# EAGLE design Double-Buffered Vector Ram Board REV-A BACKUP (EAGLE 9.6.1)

## Sheet 1 of 4: Vector Ram Control
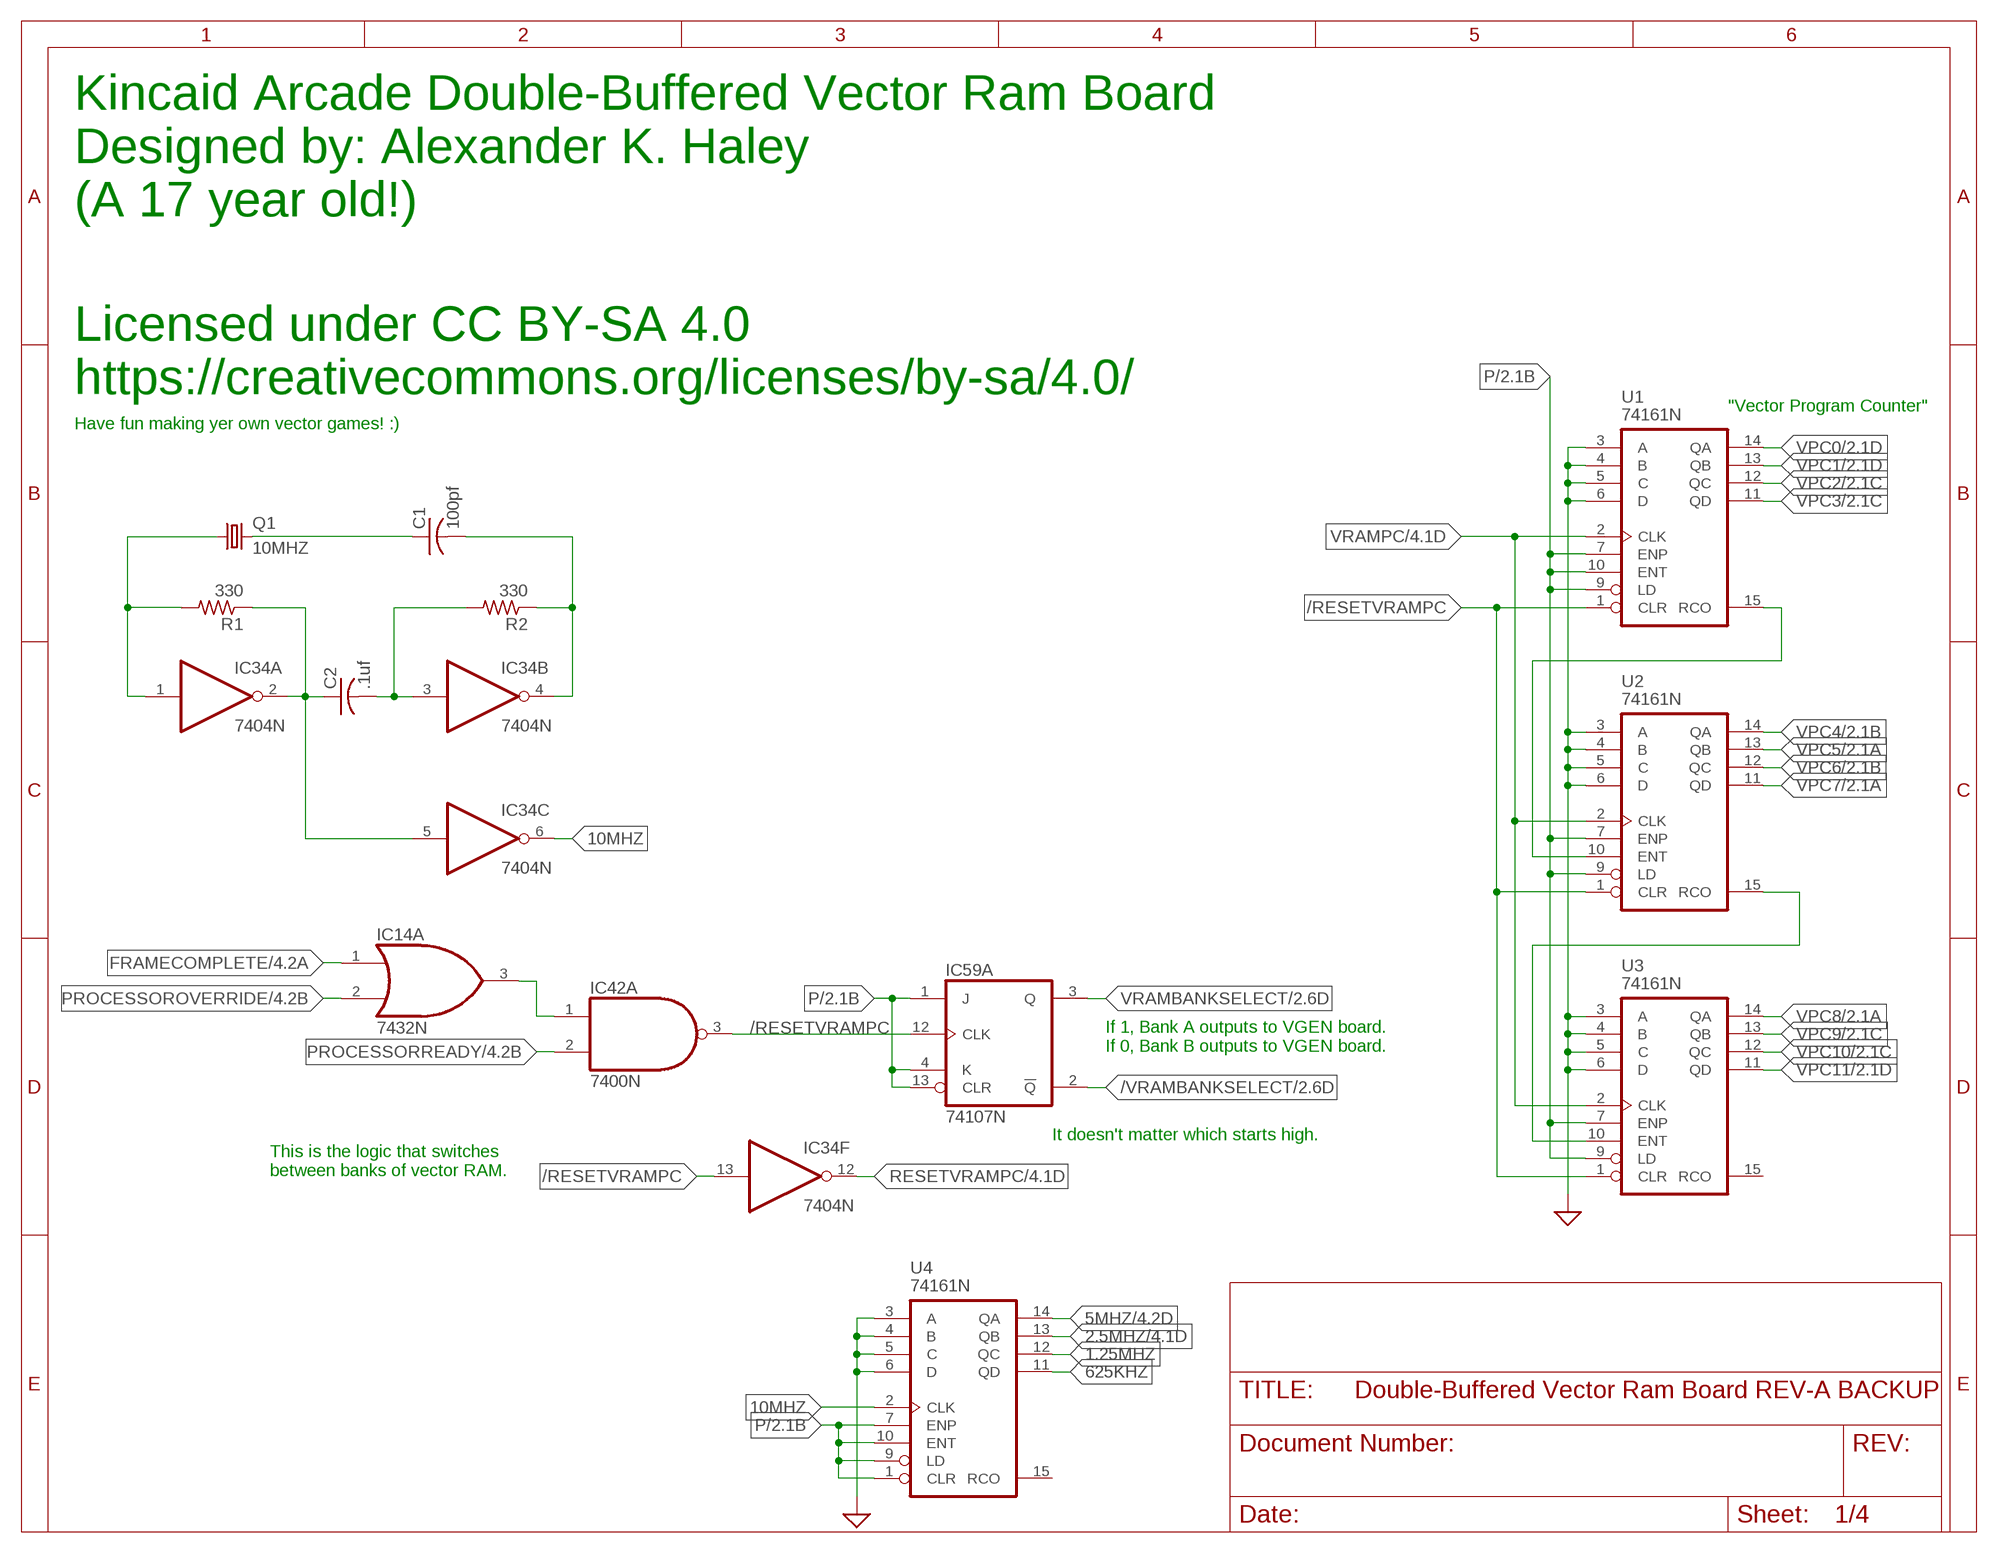
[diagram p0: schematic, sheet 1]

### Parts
C1  100pf  C-US025-030X050  [C025-030X050]
C2  .1uf  C-US050-050X075  [C050-050X075]
IC14  7432N  [DIL14]
IC34  7404N  [DIL14]
IC42  7400N  [DIL14]
IC59  74107N  [DIL14]
Q1  10MHZ  CRYSTALHC49S  [HC49/S]
R1  330  R-US_0207/10  [0207/10]
R2  330  R-US_0207/10  [0207/10]
U1  74161N  [DIL16]
U2  74161N  [DIL16]
U3  74161N  [DIL16]
U4  74161N  [DIL16]

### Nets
1.25MHZ: U4.12(QC)
2.5MHZ: U4.13(QB) ; also sheet 4
5MHZ: U4.14(QA) ; also sheet 4
10MHZ: IC34.6(C:O) U4.2(CLK)
625KHZ: U4.11(QD)
/RESETVRAMPC: IC34.13(F:I) IC42.3(A:O) IC59.12(A:CLK) U1.1(CLR) U2.1(CLR) U3.1(CLR)
/VRAMBANKSELECT: IC59.2(A:!Q) ; also sheet 2,3
FRAMECOMPLETE: IC14.1(A:I0) ; also sheet 4
GND: U1.3(A) U1.4(B) U1.5(C) U1.6(D) U2.3(A) U2.4(B) U2.5(C) U2.6(D) U3.3(A) U3.4(B) U3.5(C) U3.6(D) U4.3(A) U4.4(B) U4.5(C) U4.6(D) ; supply symbol labelled SUP ; also sheet 2,3,4
N$2: IC14.3(A:O) IC42.1(A:I0)
N$5: U2.15(RCO) U3.10(ENT)
N$6: U1.15(RCO) U2.10(ENT)
N$48: IC34.1(A:I) Q1.1 R1.2
N$52: C2.1 IC34.2(A:O) IC34.5(C:I) R1.1
N$61: C2.2 IC34.3(B:I) R2.2
N$69: C1.1 Q1.2
N$74: C1.2 IC34.4(B:O) R2.1
P: IC59.1(A:J) IC59.4(A:K) IC59.13(A:CLR) U1.7(ENP) U1.9(LD) U1.10(ENT) U2.7(ENP) U2.9(LD) U3.7(ENP) U3.9(LD) U4.1(CLR) U4.7(ENP) U4.9(LD) U4.10(ENT) ; also sheet 2,3,4
PROCESSOROVERRIDE: IC14.2(A:I1) ; also sheet 4
PROCESSORREADY: IC42.2(A:I1) ; also sheet 4
RESETVRAMPC: IC34.12(F:O) ; also sheet 4
VPC0: U1.14(QA) ; also sheet 2,3
VPC1: U1.13(QB) ; also sheet 2,3
VPC2: U1.12(QC) ; also sheet 2,3
VPC3: U1.11(QD) ; also sheet 2,3
VPC4: U2.14(QA) ; also sheet 2,3
VPC5: U2.13(QB) ; also sheet 2,3
VPC6: U2.12(QC) ; also sheet 2,3
VPC7: U2.11(QD) ; also sheet 2,3
VPC8: U3.14(QA) ; also sheet 2,3
VPC9: U3.13(QB) ; also sheet 2,3
VPC10: U3.12(QC) ; also sheet 2,3
VPC11: U3.11(QD) ; also sheet 2,3
VRAMBANKSELECT: IC59.3(A:Q) ; also sheet 2,3
VRAMPC: U1.2(CLK) U2.2(CLK) U3.2(CLK) ; also sheet 4
Unconnected: U3.15(RCO) U4.15(RCO)

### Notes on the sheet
- Kincaid Arcade Double-Buffered Vector Ram Board
- Designed by: Alexander K. Haley
- (A 17 year old!)
- Licensed under CC BY-SA 4.0
- https://creativecommons.org/licenses/by-sa/4.0/
- "Vector Program Counter"
- Have fun making yer own vector games! :)
- If 1, Bank A outputs to VGEN board.
  If 0, Bank B outputs to VGEN board.
- It doesn't matter which starts high.
- This is the logic that switches 
  between banks of vector RAM.

## Sheet 2 of 4: Vector Ram Bank A
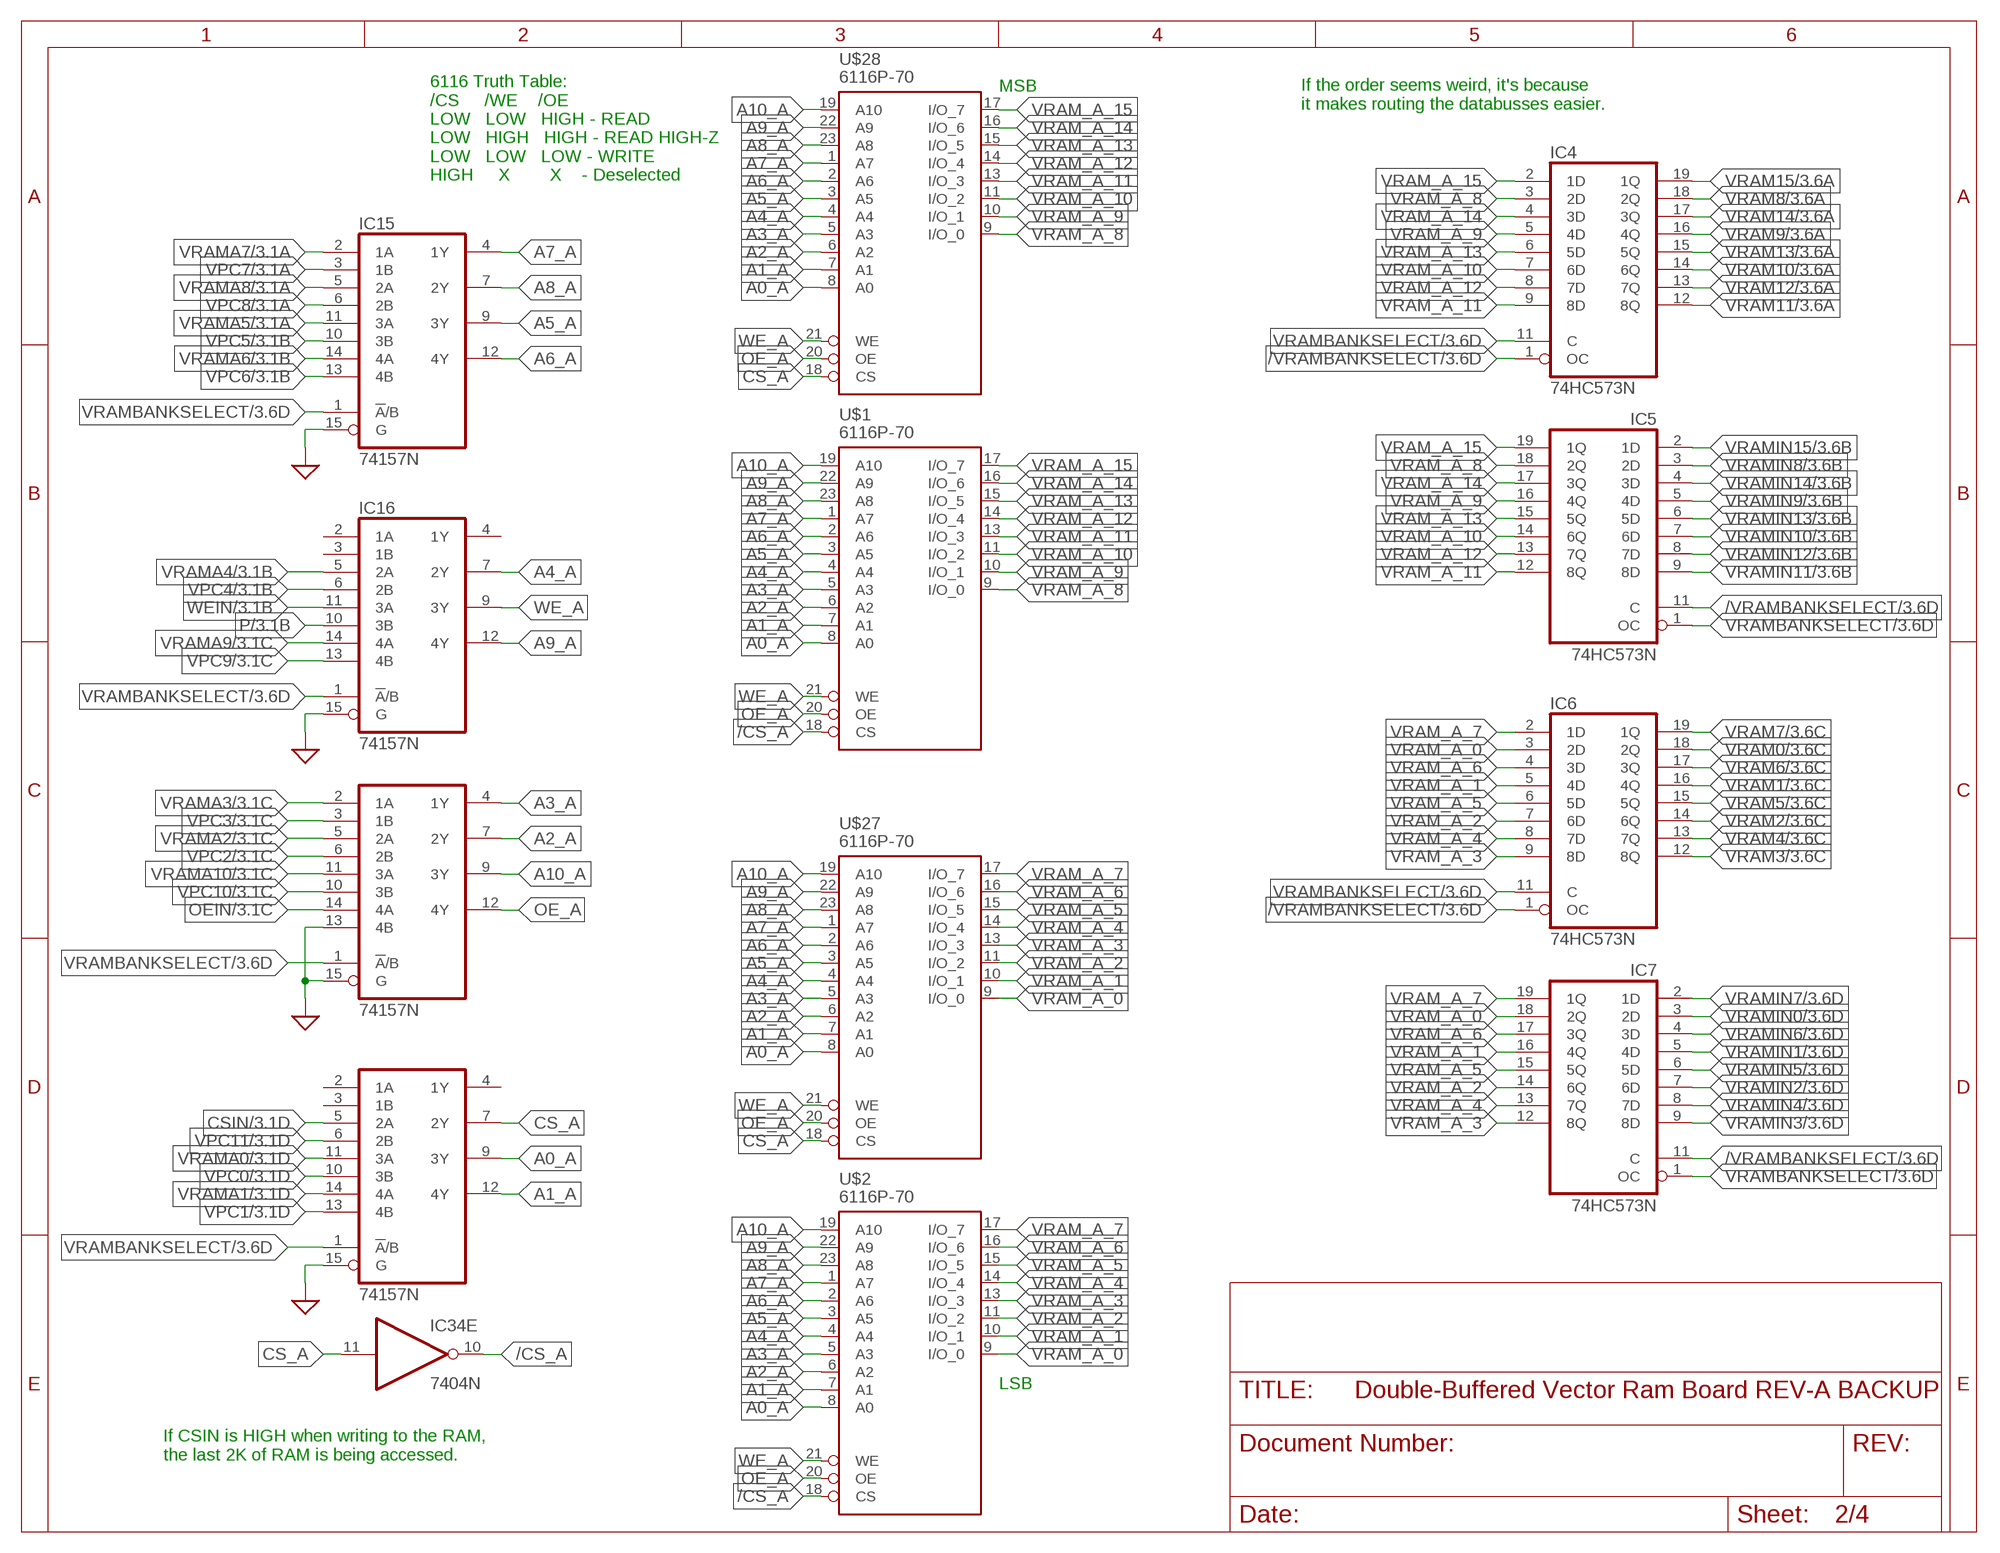
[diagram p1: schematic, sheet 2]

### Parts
IC4  74HC573N  [DIL20]
IC5  74HC573N  [DIL20]
IC6  74HC573N  [DIL20]
IC7  74HC573N  [DIL20]
IC15  74157N  [DIL16]
IC16  74157N  [DIL16]
IC17  74157N  [DIL16]
IC18  74157N  [DIL16]
U$1  6116P-70  DS1220AB/AD  [DIL24]
U$2  6116P-70  DS1220AB/AD  [DIL24]
U$27  6116P-70  [DIL24]
U$28  6116P-70  [DIL24]

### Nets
/CS_A: IC34.10(E:O) U$1.18(CS) U$2.18(CS)
/VRAMBANKSELECT: IC4.1(OC) IC5.11(C) IC6.1(OC) IC7.11(C) ; also sheet 1,3
A0_A: IC18.9(3Y) U$1.8(A0) U$2.8(A0) U$27.8(A0) U$28.8(A0)
A1_A: IC18.12(4Y) U$1.7(A1) U$2.7(A1) U$27.7(A1) U$28.7(A1)
A2_A: IC17.7(2Y) U$1.6(A2) U$2.6(A2) U$27.6(A2) U$28.6(A2)
A3_A: IC17.4(1Y) U$1.5(A3) U$2.5(A3) U$27.5(A3) U$28.5(A3)
A4_A: IC16.7(2Y) U$1.4(A4) U$2.4(A4) U$27.4(A4) U$28.4(A4)
A5_A: IC15.9(3Y) U$1.3(A5) U$2.3(A5) U$27.3(A5) U$28.3(A5)
A6_A: IC15.12(4Y) U$1.2(A6) U$2.2(A6) U$27.2(A6) U$28.2(A6)
A7_A: IC15.4(1Y) U$1.1(A7) U$2.1(A7) U$27.1(A7) U$28.1(A7)
A8_A: IC15.7(2Y) U$1.23(A8) U$2.23(A8) U$27.23(A8) U$28.23(A8)
A9_A: IC16.12(4Y) U$1.22(A9) U$2.22(A9) U$27.22(A9) U$28.22(A9)
A10_A: IC17.9(3Y) U$1.19(A10) U$2.19(A10) U$27.19(A10) U$28.19(A10)
CS_A: IC18.7(2Y) IC34.11(E:I) U$27.18(CS) U$28.18(CS)
CSIN: IC18.5(2A) ; also sheet 3,4
GND: IC15.15(G) IC16.15(G) IC17.13(4B) IC17.15(G) IC18.15(G) ; supply symbol labelled SUP ; also sheet 1,3,4
OE_A: IC17.12(4Y) U$1.20(OE) U$2.20(OE) U$27.20(OE) U$28.20(OE)
OEIN: IC17.14(4A) ; also sheet 3,4
P: IC16.10(3B) ; also sheet 1,3,4
VPC0: IC18.10(3B) ; also sheet 1,3
VPC1: IC18.13(4B) ; also sheet 1,3
VPC2: IC17.6(2B) ; also sheet 1,3
VPC3: IC17.3(1B) ; also sheet 1,3
VPC4: IC16.6(2B) ; also sheet 1,3
VPC5: IC15.10(3B) ; also sheet 1,3
VPC6: IC15.13(4B) ; also sheet 1,3
VPC7: IC15.3(1B) ; also sheet 1,3
VPC8: IC15.6(2B) ; also sheet 1,3
VPC9: IC16.13(4B) ; also sheet 1,3
VPC10: IC17.10(3B) ; also sheet 1,3
VPC11: IC18.6(2B) ; also sheet 1,3
VRAM0: IC6.18(2Q) ; also sheet 3,4
VRAM1: IC6.16(4Q) ; also sheet 3,4
VRAM2: IC6.14(6Q) ; also sheet 3,4
VRAM3: IC6.12(8Q) ; also sheet 3,4
VRAM4: IC6.13(7Q) ; also sheet 3,4
VRAM5: IC6.15(5Q) ; also sheet 3,4
VRAM6: IC6.17(3Q) ; also sheet 3,4
VRAM7: IC6.19(1Q) ; also sheet 3,4
VRAM8: IC4.18(2Q) ; also sheet 3,4
VRAM9: IC4.16(4Q) ; also sheet 3,4
VRAM10: IC4.14(6Q) ; also sheet 3,4
VRAM11: IC4.12(8Q) ; also sheet 3,4
VRAM12: IC4.13(7Q) ; also sheet 3,4
VRAM13: IC4.15(5Q) ; also sheet 3,4
VRAM14: IC4.17(3Q) ; also sheet 3,4
VRAM15: IC4.19(1Q) ; also sheet 3,4
VRAM_A_0: IC6.3(2D) IC7.18(2Q) U$2.9(I/O_0) U$27.9(I/O_0)
VRAM_A_1: IC6.5(4D) IC7.16(4Q) U$2.10(I/O_1) U$27.10(I/O_1)
VRAM_A_2: IC6.7(6D) IC7.14(6Q) U$2.11(I/O_2) U$27.11(I/O_2)
VRAM_A_3: IC6.9(8D) IC7.12(8Q) U$2.13(I/O_3) U$27.13(I/O_3)
VRAM_A_4: IC6.8(7D) IC7.13(7Q) U$2.14(I/O_4) U$27.14(I/O_4)
VRAM_A_5: IC6.6(5D) IC7.15(5Q) U$2.15(I/O_5) U$27.15(I/O_5)
VRAM_A_6: IC6.4(3D) IC7.17(3Q) U$2.16(I/O_6) U$27.16(I/O_6)
VRAM_A_7: IC6.2(1D) IC7.19(1Q) U$2.17(I/O_7) U$27.17(I/O_7)
VRAM_A_8: IC4.3(2D) IC5.18(2Q) U$1.9(I/O_0) U$28.9(I/O_0)
VRAM_A_9: IC4.5(4D) IC5.16(4Q) U$1.10(I/O_1) U$28.10(I/O_1)
VRAM_A_10: IC4.7(6D) IC5.14(6Q) U$1.11(I/O_2) U$28.11(I/O_2)
VRAM_A_11: IC4.9(8D) IC5.12(8Q) U$1.13(I/O_3) U$28.13(I/O_3)
VRAM_A_12: IC4.8(7D) IC5.13(7Q) U$1.14(I/O_4) U$28.14(I/O_4)
VRAM_A_13: IC4.6(5D) IC5.15(5Q) U$1.15(I/O_5) U$28.15(I/O_5)
VRAM_A_14: IC4.4(3D) IC5.17(3Q) U$1.16(I/O_6) U$28.16(I/O_6)
VRAM_A_15: IC4.2(1D) IC5.19(1Q) U$1.17(I/O_7) U$28.17(I/O_7)
VRAMA0: IC18.11(3A) ; also sheet 3,4
VRAMA1: IC18.14(4A) ; also sheet 3,4
VRAMA2: IC17.5(2A) ; also sheet 3,4
VRAMA3: IC17.2(1A) ; also sheet 3,4
VRAMA4: IC16.5(2A) ; also sheet 3,4
VRAMA5: IC15.11(3A) ; also sheet 3,4
VRAMA6: IC15.14(4A) ; also sheet 3,4
VRAMA7: IC15.2(1A) ; also sheet 3,4
VRAMA8: IC15.5(2A) ; also sheet 3,4
VRAMA9: IC16.14(4A) ; also sheet 3,4
VRAMA10: IC17.11(3A) ; also sheet 3,4
VRAMBANKSELECT: IC4.11(C) IC5.1(OC) IC6.11(C) IC7.1(OC) IC15.1(!A!/B) IC16.1(!A!/B) IC17.1(!A!/B) IC18.1(!A!/B) ; also sheet 1,3
VRAMIN0: IC7.3(2D) ; also sheet 3,4
VRAMIN1: IC7.5(4D) ; also sheet 3,4
VRAMIN2: IC7.7(6D) ; also sheet 3,4
VRAMIN3: IC7.9(8D) ; also sheet 3,4
VRAMIN4: IC7.8(7D) ; also sheet 3,4
VRAMIN5: IC7.6(5D) ; also sheet 3,4
VRAMIN6: IC7.4(3D) ; also sheet 3,4
VRAMIN7: IC7.2(1D) ; also sheet 3,4
VRAMIN8: IC5.3(2D) ; also sheet 3,4
VRAMIN9: IC5.5(4D) ; also sheet 3,4
VRAMIN10: IC5.7(6D) ; also sheet 3,4
VRAMIN11: IC5.9(8D) ; also sheet 3,4
VRAMIN12: IC5.8(7D) ; also sheet 3,4
VRAMIN13: IC5.6(5D) ; also sheet 3,4
VRAMIN14: IC5.4(3D) ; also sheet 3,4
VRAMIN15: IC5.2(1D) ; also sheet 3,4
WE_A: IC16.9(3Y) U$1.21(WE) U$2.21(WE) U$27.21(WE) U$28.21(WE)
WEIN: IC16.11(3A) ; also sheet 3,4
Unconnected: IC16.2(1A) IC16.3(1B) IC16.4(1Y) IC18.2(1A) IC18.3(1B) IC18.4(1Y)

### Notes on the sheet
- MSB
- If the order seems weird, it's because
  it makes routing the databusses easier.
- 6116 Truth Table:
  /CS     /WE    /OE
  LOW   LOW   HIGH - READ
  LOW   HIGH   HIGH - READ HIGH-Z
  LOW   LOW   LOW - WRITE
  HIGH     X        X    - Deselected
- LSB
- If CSIN is HIGH when writing to the RAM, 
  the last 2K of RAM is being accessed.

## Sheet 3 of 4: Vector Ram Bank B
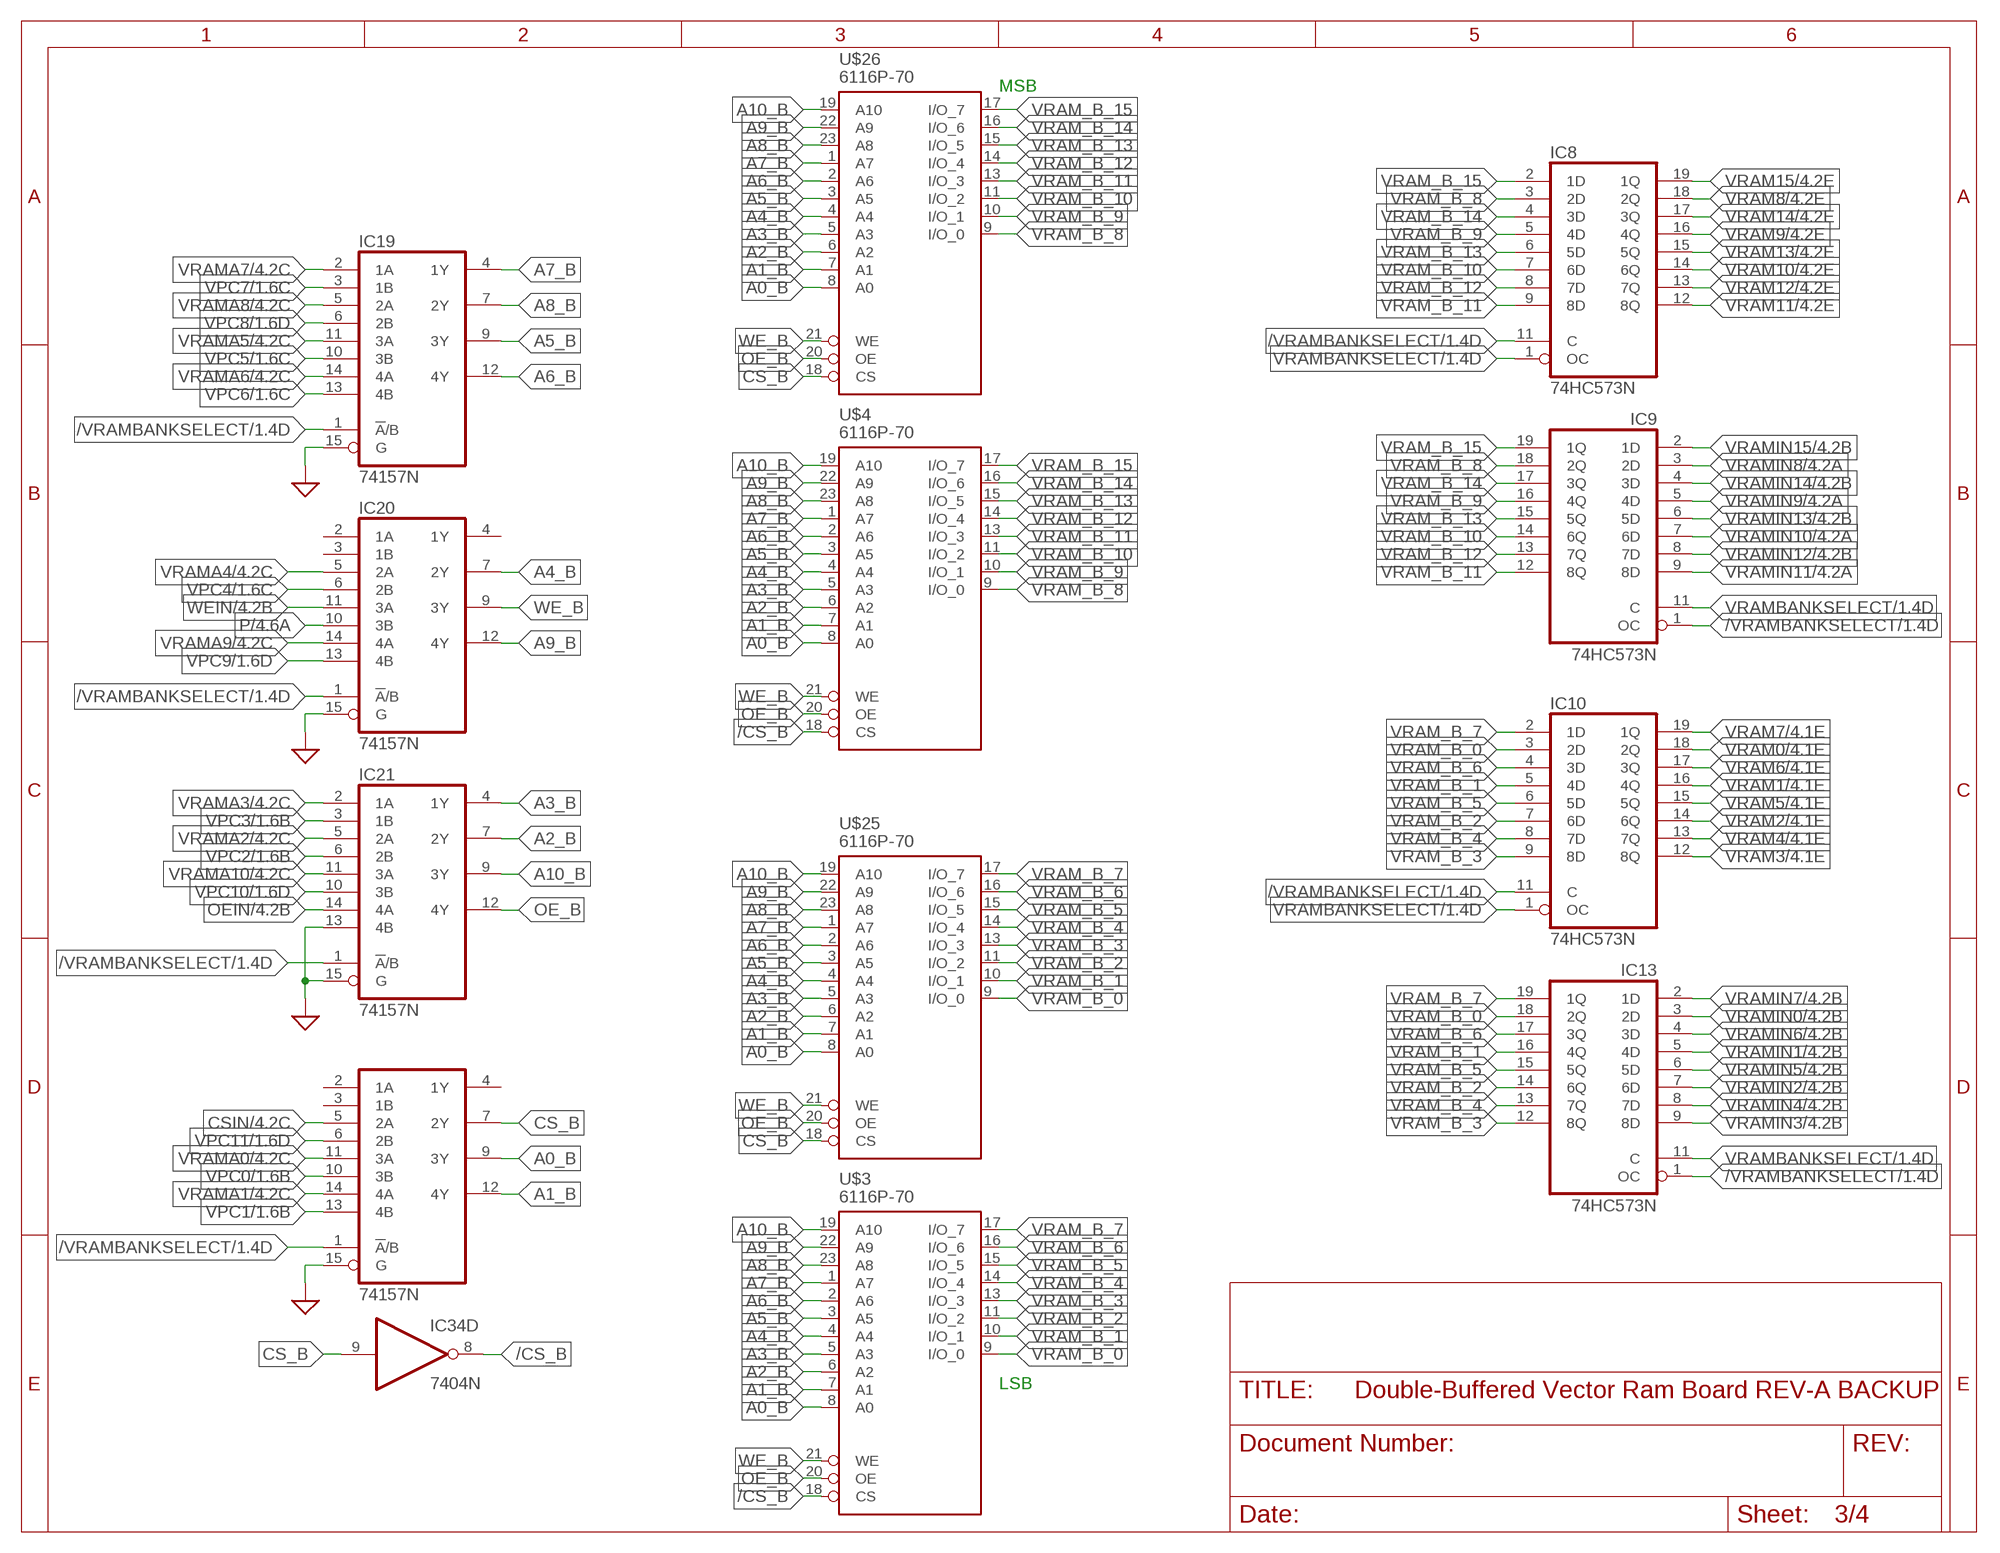
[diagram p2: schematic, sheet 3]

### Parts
IC8  74HC573N  [DIL20]
IC9  74HC573N  [DIL20]
IC10  74HC573N  [DIL20]
IC13  74HC573N  [DIL20]
IC19  74157N  [DIL16]
IC20  74157N  [DIL16]
IC21  74157N  [DIL16]
IC22  74157N  [DIL16]
U$3  6116P-70  DS1220AB/AD  [DIL24]
U$4  6116P-70  DS1220AB/AD  [DIL24]
U$25  6116P-70  [DIL24]
U$26  6116P-70  [DIL24]

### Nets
/CS_B: IC34.8(D:O) U$3.18(CS) U$4.18(CS)
/VRAMBANKSELECT: IC8.11(C) IC9.1(OC) IC10.11(C) IC13.1(OC) IC19.1(!A!/B) IC20.1(!A!/B) IC21.1(!A!/B) IC22.1(!A!/B) ; also sheet 1,2
A0_B: IC22.9(3Y) U$3.8(A0) U$4.8(A0) U$25.8(A0) U$26.8(A0)
A1_B: IC22.12(4Y) U$3.7(A1) U$4.7(A1) U$25.7(A1) U$26.7(A1)
A2_B: IC21.7(2Y) U$3.6(A2) U$4.6(A2) U$25.6(A2) U$26.6(A2)
A3_B: IC21.4(1Y) U$3.5(A3) U$4.5(A3) U$25.5(A3) U$26.5(A3)
A4_B: IC20.7(2Y) U$3.4(A4) U$4.4(A4) U$25.4(A4) U$26.4(A4)
A5_B: IC19.9(3Y) U$3.3(A5) U$4.3(A5) U$25.3(A5) U$26.3(A5)
A6_B: IC19.12(4Y) U$3.2(A6) U$4.2(A6) U$25.2(A6) U$26.2(A6)
A7_B: IC19.4(1Y) U$3.1(A7) U$4.1(A7) U$25.1(A7) U$26.1(A7)
A8_B: IC19.7(2Y) U$3.23(A8) U$4.23(A8) U$25.23(A8) U$26.23(A8)
A9_B: IC20.12(4Y) U$3.22(A9) U$4.22(A9) U$25.22(A9) U$26.22(A9)
A10_B: IC21.9(3Y) U$3.19(A10) U$4.19(A10) U$25.19(A10) U$26.19(A10)
CS_B: IC22.7(2Y) IC34.9(D:I) U$25.18(CS) U$26.18(CS)
CSIN: IC22.5(2A) ; also sheet 2,4
GND: IC19.15(G) IC20.15(G) IC21.13(4B) IC21.15(G) IC22.15(G) ; supply symbol labelled SUP ; also sheet 1,2,4
OE_B: IC21.12(4Y) U$3.20(OE) U$4.20(OE) U$25.20(OE) U$26.20(OE)
OEIN: IC21.14(4A) ; also sheet 2,4
P: IC20.10(3B) ; also sheet 1,2,4
VPC0: IC22.10(3B) ; also sheet 1,2
VPC1: IC22.13(4B) ; also sheet 1,2
VPC2: IC21.6(2B) ; also sheet 1,2
VPC3: IC21.3(1B) ; also sheet 1,2
VPC4: IC20.6(2B) ; also sheet 1,2
VPC5: IC19.10(3B) ; also sheet 1,2
VPC6: IC19.13(4B) ; also sheet 1,2
VPC7: IC19.3(1B) ; also sheet 1,2
VPC8: IC19.6(2B) ; also sheet 1,2
VPC9: IC20.13(4B) ; also sheet 1,2
VPC10: IC21.10(3B) ; also sheet 1,2
VPC11: IC22.6(2B) ; also sheet 1,2
VRAM0: IC10.18(2Q) ; also sheet 2,4
VRAM1: IC10.16(4Q) ; also sheet 2,4
VRAM2: IC10.14(6Q) ; also sheet 2,4
VRAM3: IC10.12(8Q) ; also sheet 2,4
VRAM4: IC10.13(7Q) ; also sheet 2,4
VRAM5: IC10.15(5Q) ; also sheet 2,4
VRAM6: IC10.17(3Q) ; also sheet 2,4
VRAM7: IC10.19(1Q) ; also sheet 2,4
VRAM8: IC8.18(2Q) ; also sheet 2,4
VRAM9: IC8.16(4Q) ; also sheet 2,4
VRAM10: IC8.14(6Q) ; also sheet 2,4
VRAM11: IC8.12(8Q) ; also sheet 2,4
VRAM12: IC8.13(7Q) ; also sheet 2,4
VRAM13: IC8.15(5Q) ; also sheet 2,4
VRAM14: IC8.17(3Q) ; also sheet 2,4
VRAM15: IC8.19(1Q) ; also sheet 2,4
VRAM_B_0: IC10.3(2D) IC13.18(2Q) U$3.9(I/O_0) U$25.9(I/O_0)
VRAM_B_1: IC10.5(4D) IC13.16(4Q) U$3.10(I/O_1) U$25.10(I/O_1)
VRAM_B_2: IC10.7(6D) IC13.14(6Q) U$3.11(I/O_2) U$25.11(I/O_2)
VRAM_B_3: IC10.9(8D) IC13.12(8Q) U$3.13(I/O_3) U$25.13(I/O_3)
VRAM_B_4: IC10.8(7D) IC13.13(7Q) U$3.14(I/O_4) U$25.14(I/O_4)
VRAM_B_5: IC10.6(5D) IC13.15(5Q) U$3.15(I/O_5) U$25.15(I/O_5)
VRAM_B_6: IC10.4(3D) IC13.17(3Q) U$3.16(I/O_6) U$25.16(I/O_6)
VRAM_B_7: IC10.2(1D) IC13.19(1Q) U$3.17(I/O_7) U$25.17(I/O_7)
VRAM_B_8: IC8.3(2D) IC9.18(2Q) U$4.9(I/O_0) U$26.9(I/O_0)
VRAM_B_9: IC8.5(4D) IC9.16(4Q) U$4.10(I/O_1) U$26.10(I/O_1)
VRAM_B_10: IC8.7(6D) IC9.14(6Q) U$4.11(I/O_2) U$26.11(I/O_2)
VRAM_B_11: IC8.9(8D) IC9.12(8Q) U$4.13(I/O_3) U$26.13(I/O_3)
VRAM_B_12: IC8.8(7D) IC9.13(7Q) U$4.14(I/O_4) U$26.14(I/O_4)
VRAM_B_13: IC8.6(5D) IC9.15(5Q) U$4.15(I/O_5) U$26.15(I/O_5)
VRAM_B_14: IC8.4(3D) IC9.17(3Q) U$4.16(I/O_6) U$26.16(I/O_6)
VRAM_B_15: IC8.2(1D) IC9.19(1Q) U$4.17(I/O_7) U$26.17(I/O_7)
VRAMA0: IC22.11(3A) ; also sheet 2,4
VRAMA1: IC22.14(4A) ; also sheet 2,4
VRAMA2: IC21.5(2A) ; also sheet 2,4
VRAMA3: IC21.2(1A) ; also sheet 2,4
VRAMA4: IC20.5(2A) ; also sheet 2,4
VRAMA5: IC19.11(3A) ; also sheet 2,4
VRAMA6: IC19.14(4A) ; also sheet 2,4
VRAMA7: IC19.2(1A) ; also sheet 2,4
VRAMA8: IC19.5(2A) ; also sheet 2,4
VRAMA9: IC20.14(4A) ; also sheet 2,4
VRAMA10: IC21.11(3A) ; also sheet 2,4
VRAMBANKSELECT: IC8.1(OC) IC9.11(C) IC10.1(OC) IC13.11(C) ; also sheet 1,2
VRAMIN0: IC13.3(2D) ; also sheet 2,4
VRAMIN1: IC13.5(4D) ; also sheet 2,4
VRAMIN2: IC13.7(6D) ; also sheet 2,4
VRAMIN3: IC13.9(8D) ; also sheet 2,4
VRAMIN4: IC13.8(7D) ; also sheet 2,4
VRAMIN5: IC13.6(5D) ; also sheet 2,4
VRAMIN6: IC13.4(3D) ; also sheet 2,4
VRAMIN7: IC13.2(1D) ; also sheet 2,4
VRAMIN8: IC9.3(2D) ; also sheet 2,4
VRAMIN9: IC9.5(4D) ; also sheet 2,4
VRAMIN10: IC9.7(6D) ; also sheet 2,4
VRAMIN11: IC9.9(8D) ; also sheet 2,4
VRAMIN12: IC9.8(7D) ; also sheet 2,4
VRAMIN13: IC9.6(5D) ; also sheet 2,4
VRAMIN14: IC9.4(3D) ; also sheet 2,4
VRAMIN15: IC9.2(1D) ; also sheet 2,4
WE_B: IC20.9(3Y) U$3.21(WE) U$4.21(WE) U$25.21(WE) U$26.21(WE)
WEIN: IC20.11(3A) ; also sheet 2,4
Unconnected: IC20.2(1A) IC20.3(1B) IC20.4(1Y) IC22.2(1A) IC22.3(1B) IC22.4(1Y)

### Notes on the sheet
- MSB
- LSB

## Sheet 4 of 4: Connectors, Pullups, and Filter Capacitors
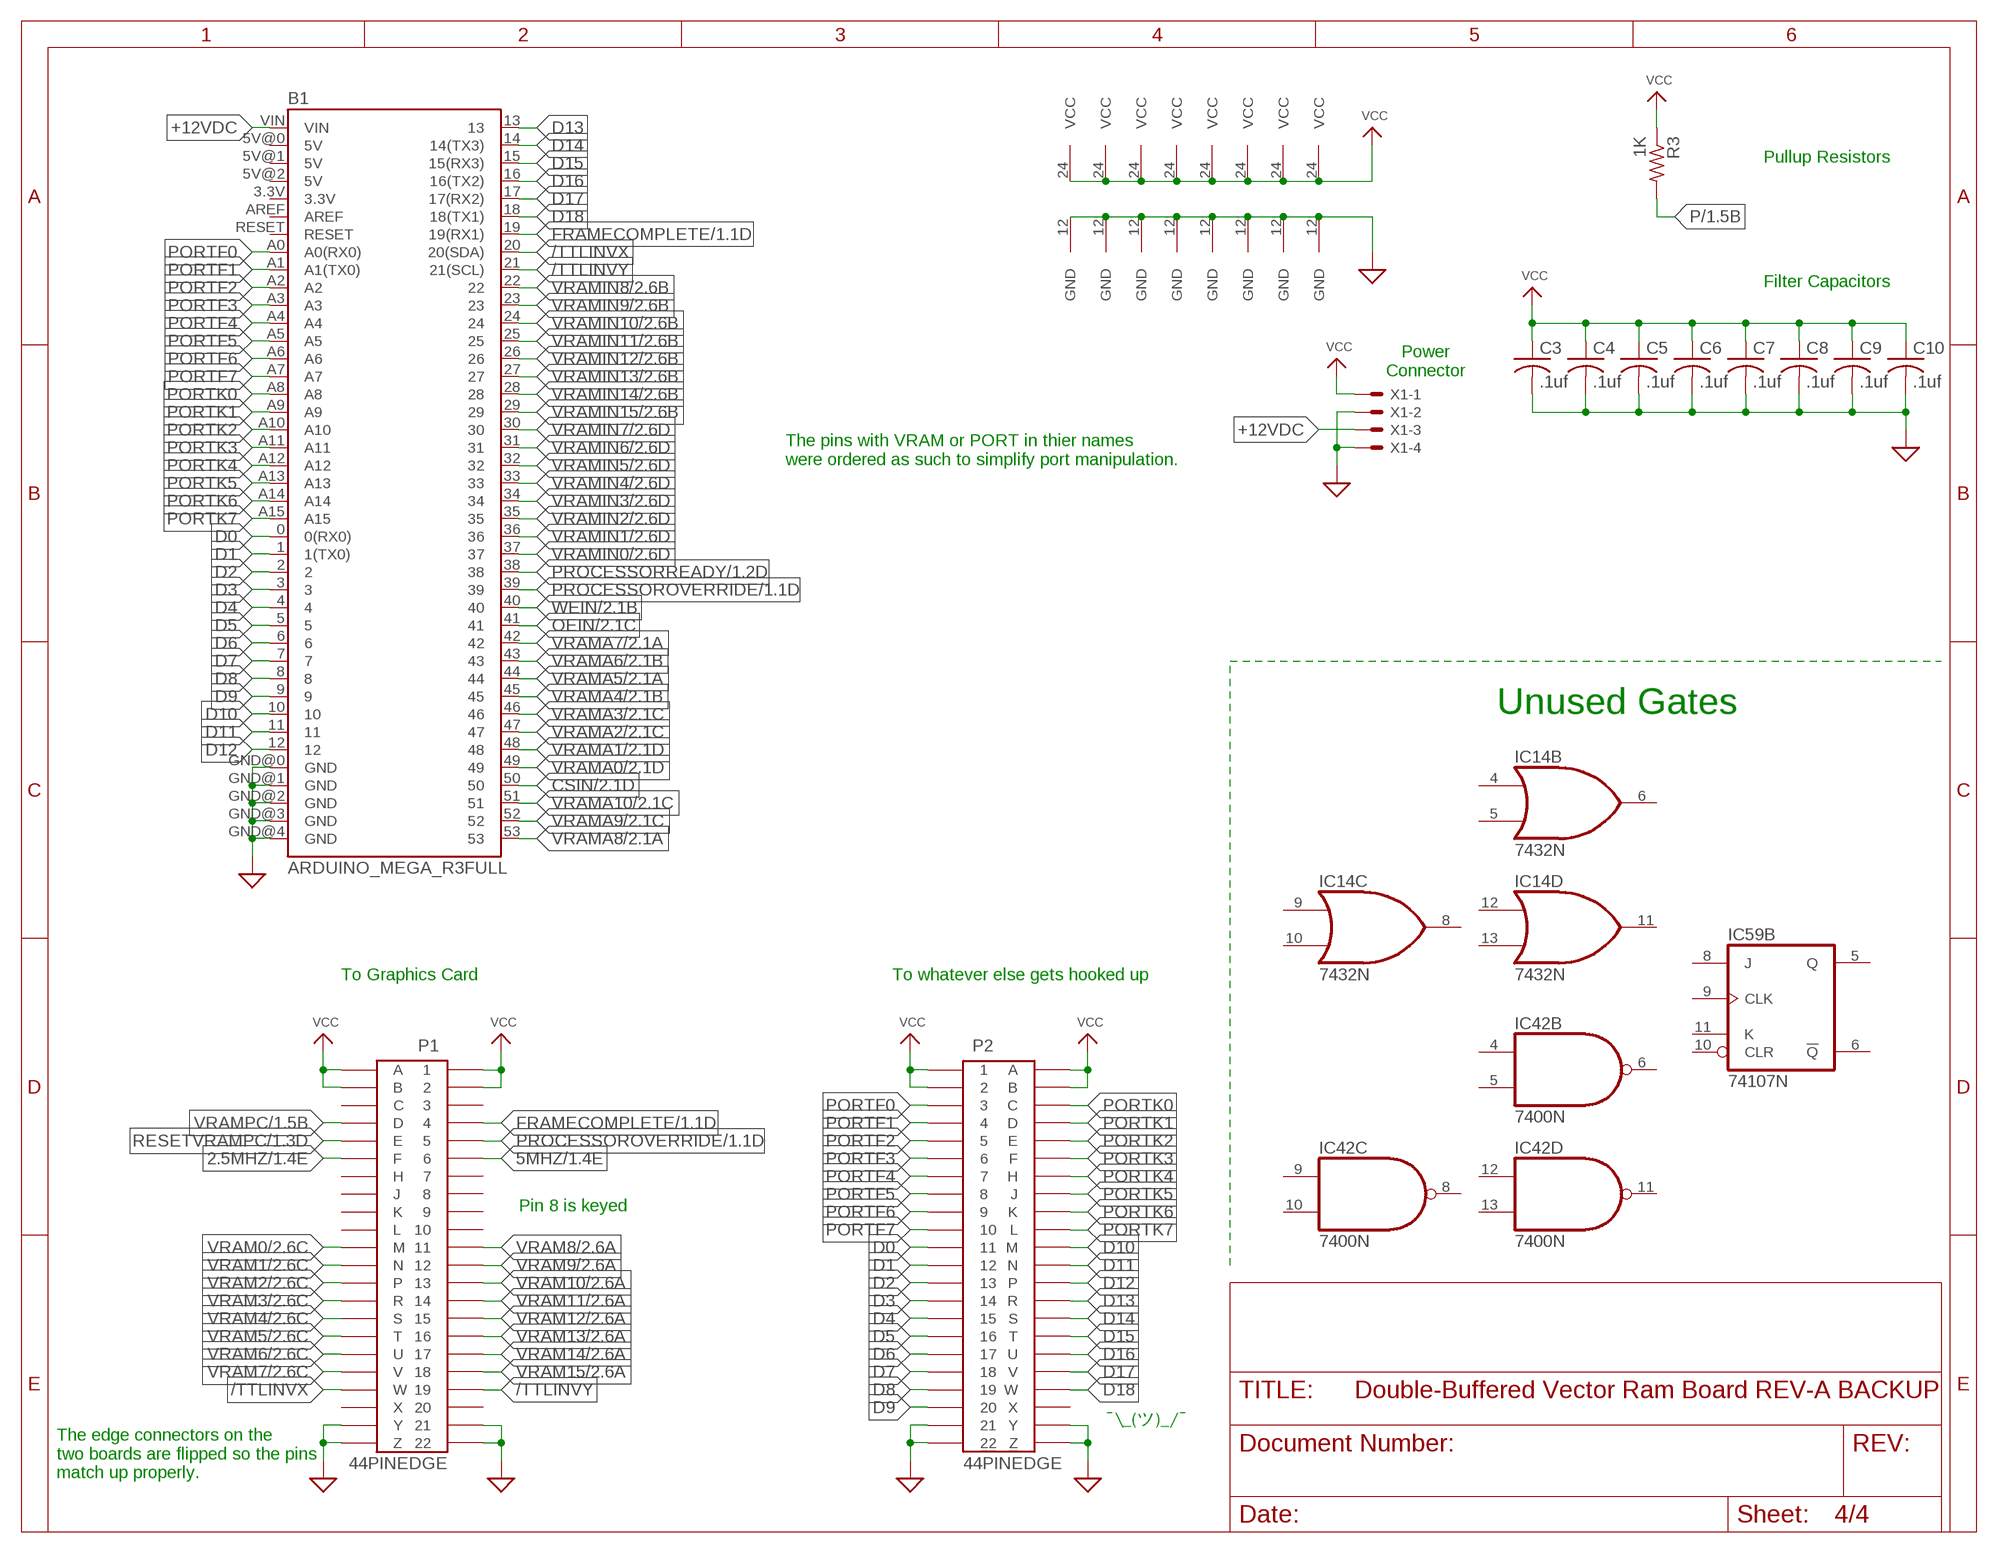
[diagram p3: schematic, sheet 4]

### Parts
B1  ARDUINO_MEGA_R3FULL  [ARDUINO_MEGA]
C3  .1uf  C-US050-025X075  [C050-025X075]
C4  .1uf  C-US050-025X075  [C050-025X075]
C5  .1uf  C-US050-025X075  [C050-025X075]
C6  .1uf  C-US050-025X075  [C050-025X075]
C7  .1uf  C-US050-025X075  [C050-025X075]
C8  .1uf  C-US050-025X075  [C050-025X075]
C9  .1uf  C-US050-025X075  [C050-025X075]
C10  .1uf  C-US050-025X075  [C050-025X075]
P1  44PINEDGE  [44PINEDGE]
P2  44PINEDGE  [44PINEDGE]
R3  1K  R-US_0207/12  [0207/12]
X1  KK-156-4  [KK-156-4]

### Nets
2.5MHZ: P1.F ; also sheet 1
5MHZ: P1.6 ; also sheet 1
+12VDC: B1.VIN X1.3
/TTLINVX: B1.20(20(SDA)) P1.W
/TTLINVY: B1.21(21(SCL)) P1.19
CSIN: B1.50 ; also sheet 2,3
D0: B1.0(0(RX0)) P2.11
D1: B1.1(1(TX0)) P2.12
D2: B1.2 P2.13
D3: B1.3 P2.14
D4: B1.4 P2.15
D5: B1.5 P2.16
D6: B1.6 P2.17
D7: B1.7 P2.18
D8: B1.8 P2.19
D9: B1.9 P2.20
D10: B1.10 P2.M
D11: B1.11 P2.N
D12: B1.12 P2.P
D13: B1.13 P2.R
D14: B1.14(14(TX3)) P2.S
D15: B1.15(15(RX3)) P2.T
D16: B1.16(16(TX2)) P2.U
D17: B1.17(17(RX2)) P2.V
D18: B1.18(18(TX1)) P2.W
FRAMECOMPLETE: B1.19(19(RX1)) P1.4 ; also sheet 1
GND: B1.GND@0(GND) B1.GND@1(GND) B1.GND@2(GND) B1.GND@3(GND) B1.GND@4(GND) C3.2 C4.2 C5.2 C6.2 C7.2 C8.2 C9.2 C10.2 P1.21 P1.22 P1.Y P1.Z P2.21 P2.22 P2.Y P2.Z U$1.12(GND) U$2.12(GND) U$3.12(GND) U$4.12(GND) U$25.12(GND) U$26.12(GND) U$27.12(GND) U$28.12(GND) X1.2 X1.4 ; supply symbol labelled SUP ; also sheet 1,2,3
OEIN: B1.41 ; also sheet 2,3
P: R3.2 ; also sheet 1,2,3
PORTF0: B1.A0(A0(RX0)) P2.3
PORTF1: B1.A1(A1(TX0)) P2.4
PORTF2: B1.A2 P2.5
PORTF3: B1.A3 P2.6
PORTF4: B1.A4 P2.7
PORTF5: B1.A5 P2.8
PORTF6: B1.A6 P2.9
PORTF7: B1.A7 P2.10
PORTK0: B1.A8 P2.C
PORTK1: B1.A9 P2.D
PORTK2: B1.A10 P2.E
PORTK3: B1.A11 P2.F
PORTK4: B1.A12 P2.H
PORTK5: B1.A13 P2.J
PORTK6: B1.A14 P2.K
PORTK7: B1.A15 P2.L
PROCESSOROVERRIDE: B1.39 P1.5 ; also sheet 1
PROCESSORREADY: B1.38 ; also sheet 1
RESETVRAMPC: P1.E ; also sheet 1
VCC: C3.1 C4.1 C5.1 C6.1 C7.1 C8.1 C9.1 C10.1 P1.1 P1.2 P1.A P1.B P2.1 P2.2 P2.A P2.B R3.1 U$1.24(VCC) U$2.24(VCC) U$3.24(VCC) U$4.24(VCC) U$25.24(VCC) U$26.24(VCC) U$27.24(VCC) U$28.24(VCC) X1.1
VRAM0: P1.M ; also sheet 2,3
VRAM1: P1.N ; also sheet 2,3
VRAM2: P1.P ; also sheet 2,3
VRAM3: P1.R ; also sheet 2,3
VRAM4: P1.S ; also sheet 2,3
VRAM5: P1.T ; also sheet 2,3
VRAM6: P1.U ; also sheet 2,3
VRAM7: P1.V ; also sheet 2,3
VRAM8: P1.11 ; also sheet 2,3
VRAM9: P1.12 ; also sheet 2,3
VRAM10: P1.13 ; also sheet 2,3
VRAM11: P1.14 ; also sheet 2,3
VRAM12: P1.15 ; also sheet 2,3
VRAM13: P1.16 ; also sheet 2,3
VRAM14: P1.17 ; also sheet 2,3
VRAM15: P1.18 ; also sheet 2,3
VRAMA0: B1.49 ; also sheet 2,3
VRAMA1: B1.48 ; also sheet 2,3
VRAMA2: B1.47 ; also sheet 2,3
VRAMA3: B1.46 ; also sheet 2,3
VRAMA4: B1.45 ; also sheet 2,3
VRAMA5: B1.44 ; also sheet 2,3
VRAMA6: B1.43 ; also sheet 2,3
VRAMA7: B1.42 ; also sheet 2,3
VRAMA8: B1.53 ; also sheet 2,3
VRAMA9: B1.52 ; also sheet 2,3
VRAMA10: B1.51 ; also sheet 2,3
VRAMIN0: B1.37 ; also sheet 2,3
VRAMIN1: B1.36 ; also sheet 2,3
VRAMIN2: B1.35 ; also sheet 2,3
VRAMIN3: B1.34 ; also sheet 2,3
VRAMIN4: B1.33 ; also sheet 2,3
VRAMIN5: B1.32 ; also sheet 2,3
VRAMIN6: B1.31 ; also sheet 2,3
VRAMIN7: B1.30 ; also sheet 2,3
VRAMIN8: B1.22 ; also sheet 2,3
VRAMIN9: B1.23 ; also sheet 2,3
VRAMIN10: B1.24 ; also sheet 2,3
VRAMIN11: B1.25 ; also sheet 2,3
VRAMIN12: B1.26 ; also sheet 2,3
VRAMIN13: B1.27 ; also sheet 2,3
VRAMIN14: B1.28 ; also sheet 2,3
VRAMIN15: B1.29 ; also sheet 2,3
VRAMPC: P1.D ; also sheet 1
WEIN: B1.40 ; also sheet 2,3
Unconnected: B1.3.3V B1.5V@0(5V) B1.5V@1(5V) B1.5V@2(5V) B1.AREF B1.RESET IC14.4(B:I0) IC14.5(B:I1) IC14.6(B:O) IC14.8(C:O) IC14.9(C:I0) IC14.10(C:I1) IC14.11(D:O) IC14.12(D:I0) IC14.13(D:I1) IC42.4(B:I0) IC42.5(B:I1) IC42.6(B:O) IC42.8(C:O) IC42.9(C:I0) IC42.10(C:I1) IC42.11(D:O) IC42.12(D:I0) IC42.13(D:I1) IC59.5(B:Q) IC59.6(B:!Q) IC59.8(B:J) IC59.9(B:CLK) IC59.10(B:CLR) IC59.11(B:K) P1.3 P1.7 P1.8 P1.9 P1.10 P1.20 P1.C P1.H P1.J P1.K P1.L P1.X P2.X

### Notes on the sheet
- Pullup Resistors
- Filter Capacitors
- Power
  Connector
- The pins with VRAM or PORT in thier names
  were ordered as such to simplify port manipulation.
- Unused Gates
- To Graphics Card | To whatever else gets hooked up
- Pin 8 is keyed
- ¯\_(ツ)_/¯
- The edge connectors on the
  two boards are flipped so the pins
  match up properly.

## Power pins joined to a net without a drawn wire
GND: IC4.10(GND) IC5.10(GND) IC6.10(GND) IC7.10(GND) IC8.10(GND) IC9.10(GND) IC10.10(GND) IC13.10(GND) IC14.7(P:GND) IC15.8(GND) IC16.8(GND) IC17.8(GND) IC18.8(GND) IC19.8(GND) IC20.8(GND) IC21.8(GND) IC22.8(GND) IC34.7(P:GND) IC42.7(P:GND) IC59.7(P:GND) U1.8(GND) U2.8(GND) U3.8(GND) U4.8(GND)
VCC: IC4.20(VCC) IC5.20(VCC) IC6.20(VCC) IC7.20(VCC) IC8.20(VCC) IC9.20(VCC) IC10.20(VCC) IC13.20(VCC) IC14.14(P:VCC) IC15.16(VCC) IC16.16(VCC) IC17.16(VCC) IC18.16(VCC) IC19.16(VCC) IC20.16(VCC) IC21.16(VCC) IC22.16(VCC) IC34.14(P:VCC) IC42.14(P:VCC) IC59.14(P:VCC) U1.16(VCC) U2.16(VCC) U3.16(VCC) U4.16(VCC)

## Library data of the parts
B1 = SparkFun-Boards:ARDUINO_MEGA_R3: Arduino Mega R3 ATmega2560 R3 compatible footprint. SparkFun Products: Arduino Mega 2560 R3
C1-C10 = rcl:C-US: CAPACITOR, American symbol; SPICEPREFIX: C
IC4-IC10 IC13 = 74xx-us:74*573: 8-bit D latch BUS DRIVER
IC14 = 74xx-us:74*32: Quad 2-input OR gate
IC15-IC22 = 74xx-us:74*157: Quadruple 2-line to 1-line data SELECTOR/MULTIPLEXER
IC34 = 74xx-us:74*04: Hex INVERTER
IC42 = 74xx-us:74*00: Quad 2-input NAND gate
IC59 = 74xx-us:74*107: Dual J-K FLIP FLOP, clear
P1 P2 = edge-156:44PINEDGE: 44 PIN EDGE CONNECTOR FOR PCB
Q1 = crystal:CRYSTAL: CRYSTAL; OC_FARNELL: 1667008; OC_NEWARK: unknown
R1 R2 = rcl:R-US_: RESISTOR, American symbol; SPICEPREFIX: R
R3 = resistor:R-US_: RESISTOR, American symbol
U1-U4 = oldchips:74*161: Synchronous 4-bit COUNTER with direct clear
U$1-U$4 = OLD AND OBSOLETE ARCADE PARTS:DS1220AB/AD: A nonvolatile SRAM chip, pin compatible with the 6116, 2716, or any other device that uses this standard.
U$25-U$28 = OLD AND OBSOLETE ARCADE PARTS:6116P-70: 6116P-70, 16K SRAM
X1 = con-molex:KK-156-4: KK 156 HEADER Source: http://www.molex.com/pdm_docs/sd/026604100_sd.pdf; MF: MOLEX; OC_FARNELL: unknown; OC_NEWARK: unknown

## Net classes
0 default: width 0.406 mm, clearance 0.406 mm

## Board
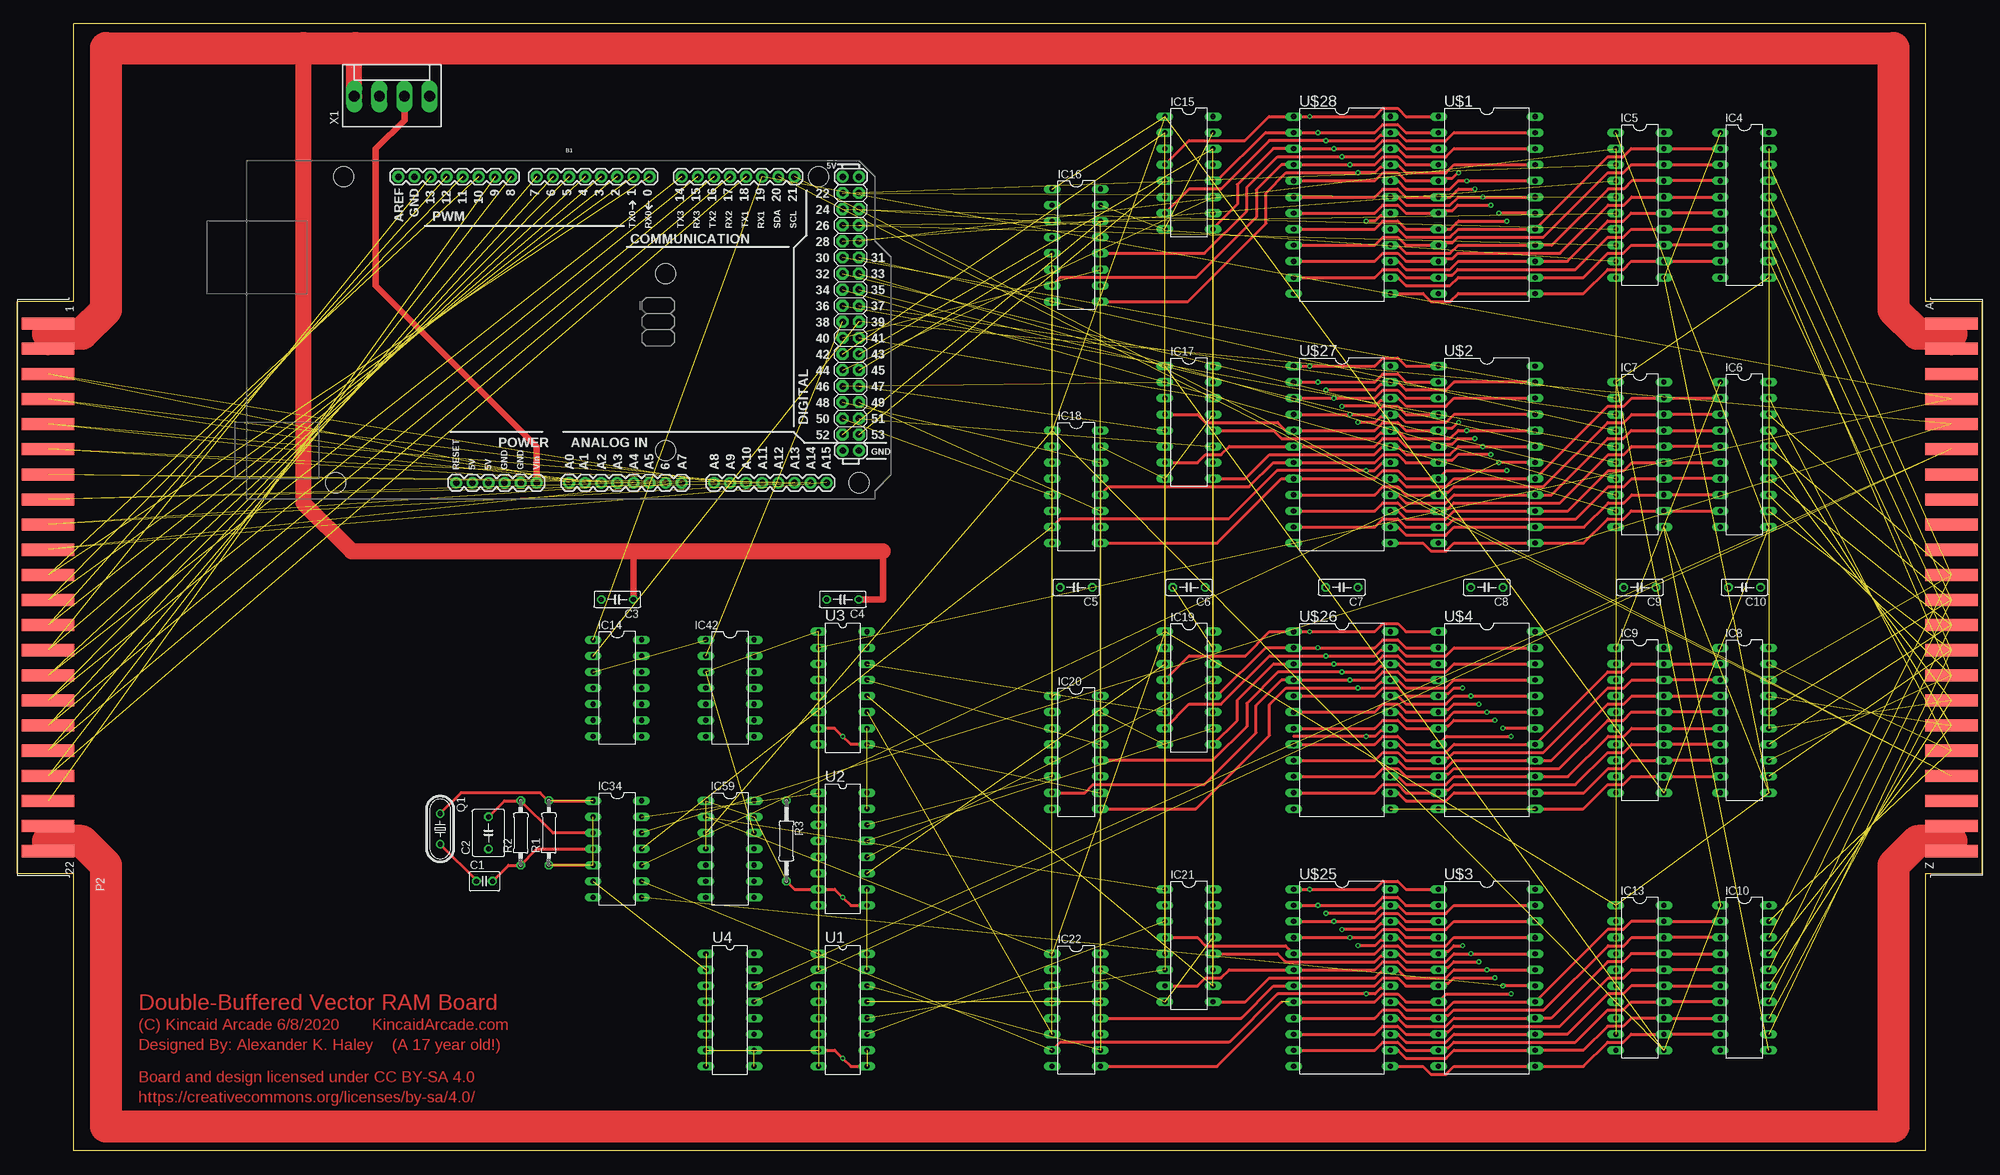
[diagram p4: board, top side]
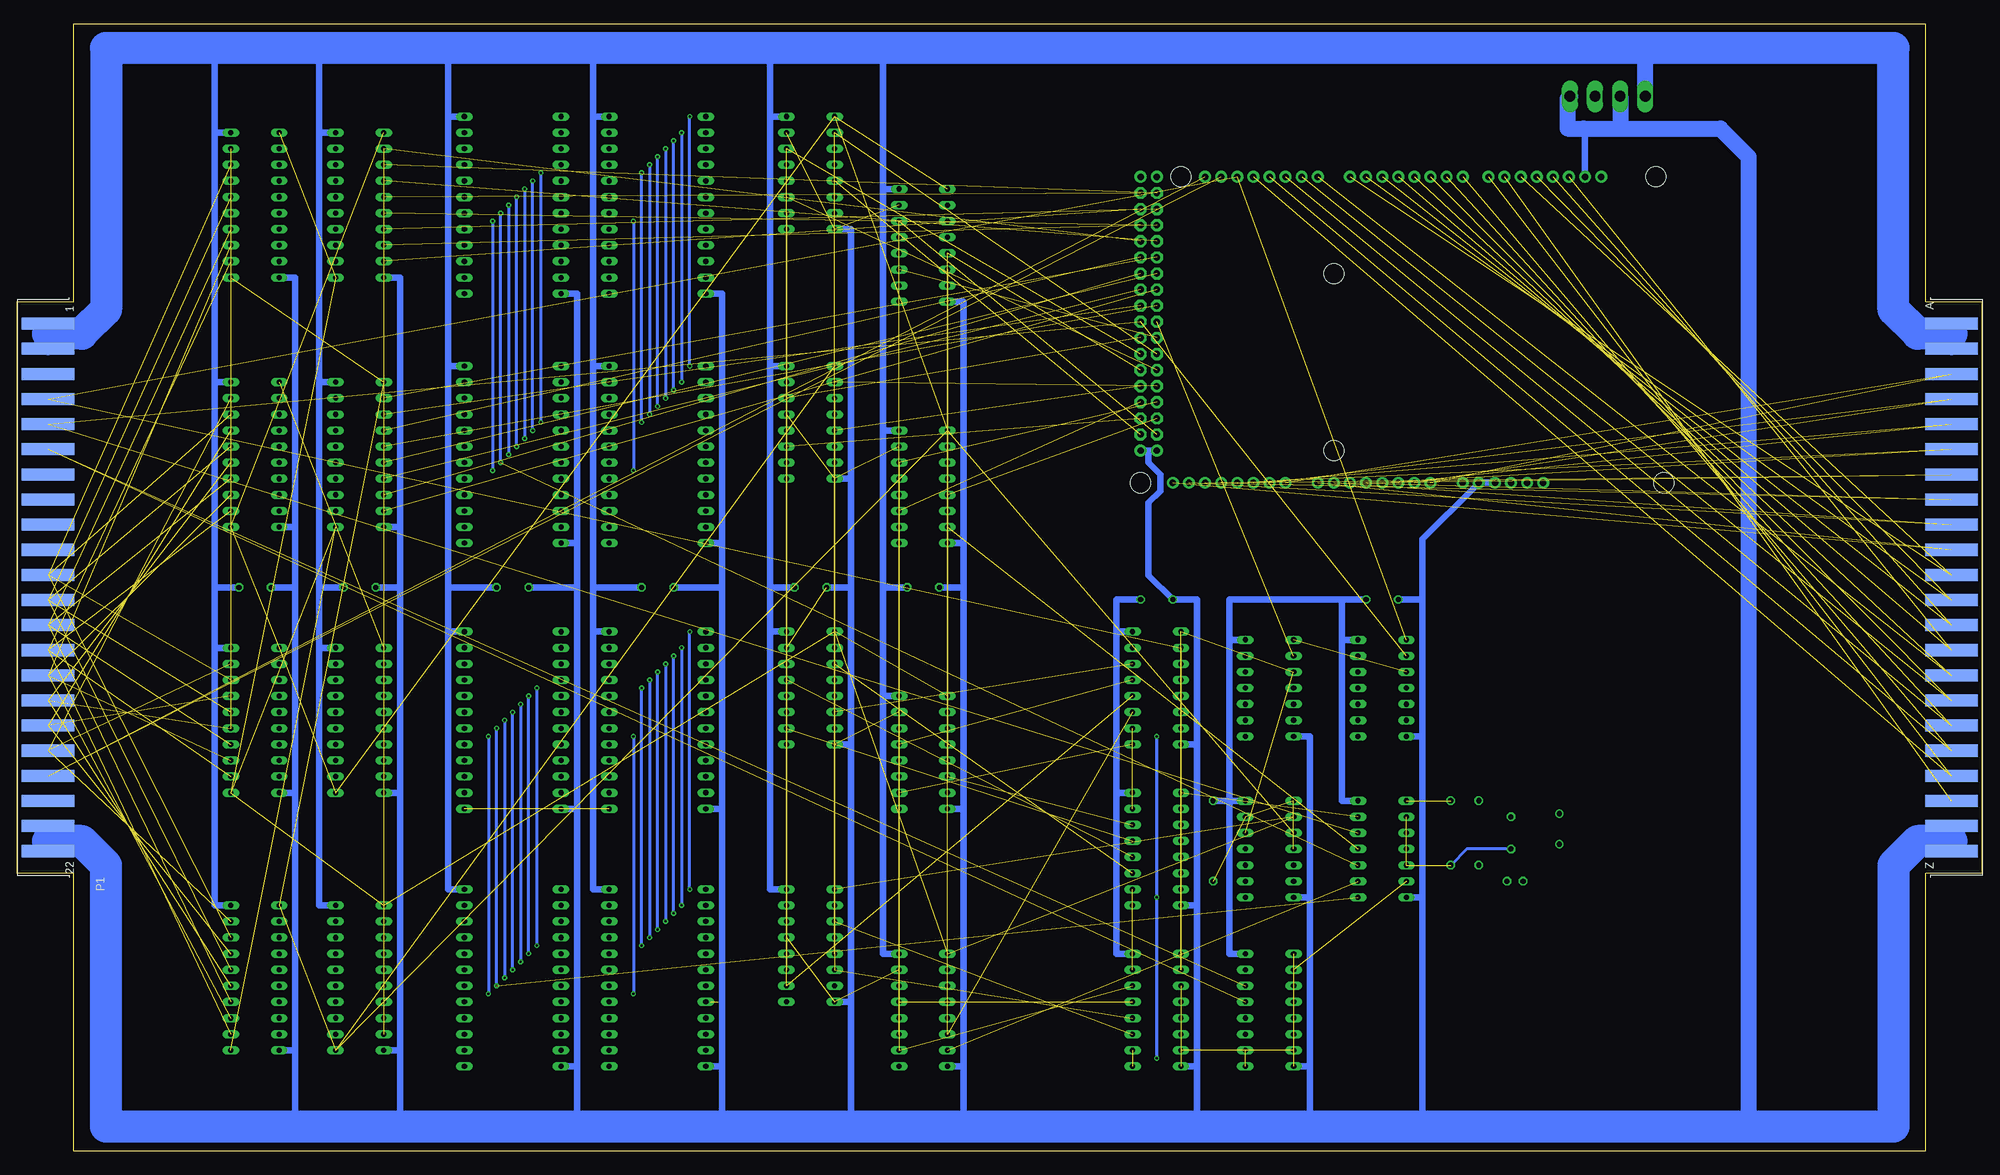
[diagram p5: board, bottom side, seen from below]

Size 309.88 x 177.8 mm. Coordinates in mm from the lower left corner, seen from the top.
Outline: 300.99,0 300.99,43.81 309.88,43.81 309.88,133.99 300.99,133.99 300.99,177.8 300.35,177.8 8.89,177.8 8.89,176.53 8.89,133.99 0,133.99 0,43.81 8.89,43.81 8.89,0 300.99,0
Copper layers (1*16): Top 0.035mm / dielectric 1.5mm / Bottom 0.035mm
Design rules "default": minimum track width 6mil, minimum drill 0.35mm, track to track 6mil, track to pad 6mil, pad to pad 6mil, via to via 6mil, smd to smd 6mil, copper to edge 40mil, drill to drill 6mil, minimum pad ring 10mil, minimum via ring 8mil, stop-mask expansion 4mil, vias tented up to drill 0mil, thermal gap 10mil

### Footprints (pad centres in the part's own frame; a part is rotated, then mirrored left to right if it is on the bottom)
ARDUINO_MEGA = drill 1.016 pad 1.88: 0 13.97,24.13; 1 11.43,24.13; 2 8.89,24.13; 3 6.35,24.13; 3.3V -13.97,-24.13; 4 3.81,24.13; 5 1.27,24.13; 5V@0 -11.43,-24.13; 5V@1 44.45,24.13; 5V@2 46.99,24.13; 6 -1.27,24.13; 7 -3.81,24.13; 8 -7.874,24.13; 9 -10.414,24.13; 10 -12.954,24.13; 11 -15.494,24.13; 12 -18.034,24.13; 13 -20.574,24.13; 14 19.05,24.13; 15 21.59,24.13; 16 24.13,24.13; 17 26.67,24.13; 18 29.21,24.13; 19 31.75,24.13; 20 34.29,24.13; 21 36.83,24.13; A0 1.27,-24.13; A1 3.81,-24.13; A2 6.35,-24.13; A3 8.89,-24.13; A4 11.43,-24.13; A5 13.97,-24.13; A6 16.51,-24.13; A7 19.05,-24.13; A8 24.13,-24.13; A9 26.67,-24.13; A10 29.21,-24.13; A11 31.75,-24.13; A12 34.29,-24.13; A13 36.83,-24.13; A14 39.37,-24.13; A15 41.91,-24.13; AREF -25.654,24.13; GND@0 -8.89,-24.13; GND@1 -6.35,-24.13; GND@2 44.45,-19.05; GND@3 46.99,-19.05; GND@4 -23.114,24.13; RESET -16.51,-24.13; VIN -3.81,-24.13 | drill 1.016 pad 1.88 octagon: 22 44.45,21.59; 23 46.99,21.59; 24 44.45,19.05; 25 46.99,19.05; 26 44.45,16.51; 27 46.99,16.51; 28 44.45,13.97; 29 46.99,13.97; 30 44.45,11.43; 31 46.99,11.43; 32 44.45,8.89; 33 46.99,8.89; 34 44.45,6.35; 35 46.99,6.35; 36 44.45,3.81; 37 46.99,3.81; 38 44.45,1.27; 39 46.99,1.27; 40 44.45,-1.27; 41 46.99,-1.27; 42 44.45,-3.81; 43 46.99,-3.81; 44 44.45,-6.35; 45 46.99,-6.35; 46 44.45,-8.89; 47 46.99,-8.89; 48 44.45,-11.43; 49 46.99,-11.43; 50 44.45,-13.97; 51 46.99,-13.97; 52 44.45,-16.51; 53 46.99,-16.51 | hole 3.2: -34.29,24.13; -35.56,-24.13; 16.51,8.89; 16.51,-19.05; 40.64,24.13; 46.99,-24.13
C025-030X050 = drill 0.813 octagon: 1 -1.27,0; 2 1.27,0
C050-050X075 = drill 0.813 octagon: 1 -2.54,0; 2 2.54,0
C050-025X075 = drill 0.813 octagon: 1 -2.54,0; 2 2.54,0
DIL20 = drill 0.813 long: 1 -11.43,-3.81; 2 -8.89,-3.81; 3 -6.35,-3.81; 4 -3.81,-3.81; 5 -1.27,-3.81; 6 1.27,-3.81; 7 3.81,-3.81; 8 6.35,-3.81; 9 8.89,-3.81; 10 11.43,-3.81; 11 11.43,3.81; 12 8.89,3.81; 13 6.35,3.81; 14 3.81,3.81; 15 1.27,3.81; 16 -1.27,3.81; 17 -3.81,3.81; 18 -6.35,3.81; 19 -8.89,3.81; 20 -11.43,3.81
DIL14 = drill 0.813 long: 1 -7.62,-3.81; 2 -5.08,-3.81; 3 -2.54,-3.81; 4 0,-3.81; 5 2.54,-3.81; 6 5.08,-3.81; 7 7.62,-3.81; 8 7.62,3.81; 9 5.08,3.81; 10 2.54,3.81; 11 0,3.81; 12 -2.54,3.81; 13 -5.08,3.81; 14 -7.62,3.81
DIL16 = drill 0.813 long: 1 -8.89,-3.81; 2 -6.35,-3.81; 3 -3.81,-3.81; 4 -1.27,-3.81; 5 1.27,-3.81; 6 3.81,-3.81; 7 6.35,-3.81; 8 8.89,-3.81; 9 8.89,3.81; 10 6.35,3.81; 11 3.81,3.81; 12 1.27,3.81; 13 -1.27,3.81; 14 -3.81,3.81; 15 -6.35,3.81; 16 -8.89,3.81
44PINEDGE = smd 1.905 x 8.255: 1 -41.605,4.826; 2 -37.643,4.826; 3 -33.68,4.826; 4 -29.718,4.826; 5 -25.756,4.826; 6 -21.793,4.826; 7 -17.831,4.826; 8 -13.868,4.826; 9 -9.906,4.826; 10 -5.944,4.826; 11 -1.981,4.826; 12 1.981,4.826; 13 5.944,4.826; 14 9.906,4.826; 15 13.868,4.826; 16 17.831,4.826; 17 21.793,4.826; 18 25.756,4.826; 19 29.718,4.826; 20 33.68,4.826; 21 37.643,4.826; 22 41.605,4.826 | smd 1.905 x 8.255 bottom: A -41.605,4.826; B -37.643,4.826; C -33.68,4.826; D -29.718,4.826; E -25.756,4.826; F -21.793,4.826; H -17.831,4.826; J -13.868,4.826; K -9.906,4.826; L -5.944,4.826; M -1.981,4.826; N 1.981,4.826; P 5.944,4.826; R 9.906,4.826; S 13.868,4.826; T 17.831,4.826; U 21.793,4.826; V 25.756,4.826; W 29.718,4.826; X 33.68,4.826; Y 37.643,4.826; Z 41.605,4.826
HC49/S = drill 0.813: 1 -2.413,0; 2 2.413,0
0207/10 = drill 0.813 octagon: 1 -5.08,0; 2 5.08,0
0207/12 = drill 0.813 octagon: 1 -6.35,0; 2 6.35,0
DIL24 = drill 0.813 long: 1 -13.97,-7.62; 2 -11.43,-7.62; 3 -8.89,-7.62; 4 -6.35,-7.62; 5 -3.81,-7.62; 6 -1.27,-7.62; 7 1.27,-7.62; 8 3.81,-7.62; 9 6.35,-7.62; 10 8.89,-7.62; 11 11.43,-7.62; 12 13.97,-7.62; 13 13.97,7.62; 14 11.43,7.62; 15 8.89,7.62; 16 6.35,7.62; 17 3.81,7.62; 18 1.27,7.62; 19 -1.27,7.62; 20 -3.81,7.62; 21 -6.35,7.62; 22 -8.89,7.62; 23 -11.43,7.62; 24 -13.97,7.62
KK-156-4 = drill 1.7 pad 2.184 long: 1 -5.94,0; 2 -1.98,0; 3 1.98,0; 4 5.94,0

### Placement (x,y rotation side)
B1  85.72,129.54 0 top
C1  73.66,42.55 0 top
C2  74.3,50.16 90 top
C3  94.61,87 180 top
C4  130.18,87 180 top
C5  167,88.9 180 top
C6  184.79,88.9 180 top
C7  208.92,88.9 180 top
C8  231.77,88.9 180 top
C9  255.9,88.9 180 top
C10  272.41,88.9 180 top
IC4  272.41,149.22 270 top
IC5  255.9,149.22 270 top
IC6  272.41,109.86 270 top
IC7  255.9,109.86 270 top
IC8  272.41,67.94 270 top
IC9  255.9,67.94 270 top
IC10  272.41,27.3 270 top
IC13  255.9,27.3 270 top
IC14  94.61,73.03 270 top
IC15  184.79,154.31 270 top
IC16  167,142.88 270 top
IC17  184.79,114.94 270 top
IC18  167,104.78 270 top
IC19  184.79,73.03 270 top
IC20  167,62.87 270 top
IC21  184.79,32.38 270 top
IC22  167,22.23 270 top
IC34  94.61,47.62 270 top
IC42  112.39,73.03 270 top
IC59  112.39,47.62 270 top
P1  309.88,88.9 270 bottom
P2  0,88.9 270 top
Q1  66.67,50.8 270 top
R1  83.82,50.16 90 top
R2  79.38,50.16 90 top
R3  121.28,48.9 270 top
U1  130.18,22.23 270 top
U2  130.18,47.62 270 top
U3  130.18,73.03 270 top
U4  112.39,22.23 270 top
U$1  231.77,149.22 270 top
U$2  231.77,109.86 270 top
U$3  231.77,27.3 270 top
U$4  231.77,67.94 270 top
U$25  208.92,27.3 270 top
U$26  208.92,67.94 270 top
U$27  208.92,109.86 270 top
U$28  208.92,149.22 270 top
X1  59.05,166.37 0 top

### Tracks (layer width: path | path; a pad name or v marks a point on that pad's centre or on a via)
2.5MHZ  (1 unrouted)
5MHZ  (1 unrouted)
10MHZ  (1 unrouted)
+12VDC
  Top 1.016: X1.3 61.04,162.63 56.52,158.12 56.52,136.53 81.92,111.12 B1.VIN
/CS_A  (via drill 0.35)  (1 unrouted)
  Top 0.508: U$1.18 v233.68,147.96 | U$2.18 v233.68,108.58
  Bottom 0.508: v233.68,108.58 v233.68,147.96
/CS_B  (via drill 0.35)  (1 unrouted)
  Top 0.508: U$4.18 v234.31,66.67 | U$3.18 v234.31,26.04
  Bottom 0.508: v234.31,26.04 v234.31,66.67
/RESETVRAMPC  (5 unrouted)
/TTLINVX  (1 unrouted)
/TTLINVY  (1 unrouted)
/VRAMBANKSELECT  (12 unrouted)
A0_A  (via drill 0.35)
  Top 0.508: U$28.8 214.08,145.41 215.35,146.69 217.72,146.69 218.99,145.41 U$1.8 | U$1.8 224.79,145.41 | U$1.8 226.02,145.41 226.89,146.28 226.92,146.28 227.33,146.69 v234.95,146.69 | v234.95,107.31 225.43,107.31 U$2.8 218.99,106.05 217.72,107.31 215.35,107.31 214.08,106.05 U$27.8 199.39,106.05 189.23,95.89 IC18.9
  Bottom 0.508: v234.95,146.69 v234.95,107.31
A0_B  (via drill 0.35)  (1 unrouted)
  Top 0.508: U$26.8 214.08,64.14 215.35,65.41 217.72,65.41 218.99,64.14 U$4.8 225.43,65.41 v235.58,65.41 | 200.58,23.5 U$25.8 214.08,23.5 215.35,24.77 217.72,24.77 218.99,23.5 U$3.8 225.43,24.77 v235.58,24.77 | IC22.9 189.23,13.34 199.39,23.5
  Bottom 0.508: v235.58,65.41 v235.58,24.77
A1_A  (via drill 0.35)
  Top 0.508: U$28.7 214.08,147.96 215.35,149.22 217.72,149.22 218.99,147.96 U$1.7 224.56,148.36 226.33,148.36 227.2,149.22 v232.41,149.22 | v232.41,109.86 227.2,109.86 226.33,108.99 224.56,108.99 U$2.7 218.99,108.58 217.72,109.86 215.35,109.86 214.08,108.58 U$27.7 198.07,108.58 194.26,104.78 172.08,104.78 IC18.12
  Bottom 0.508: v232.41,149.22 v232.41,109.86
A1_B  (via drill 0.35)
  Top 0.508: U$26.7 214.08,66.67 215.35,67.94 217.72,67.94 218.99,66.67 U$4.7 224.56,67.08 225.7,67.08 226.56,67.94 v233.05,67.94 | v233.05,27.3 226.56,27.3 225.7,26.44 224.56,26.44 U$3.7 218.99,26.04 217.72,27.3 215.35,27.3 214.08,26.04 U$25.7 198.12,26.04 193.04,20.95 IC22.12
  Bottom 0.508: v233.05,67.94 v233.05,27.3
A2_A  (via drill 0.35)
  Top 0.508: U$28.6 214.08,150.5 215.35,151.76 217.72,151.76 218.99,150.5 U$1.6 226.02,150.5 226.89,151.36 226.92,151.36 227.33,151.76 v229.87,151.76 | v229.87,112.39 227.2,112.39 226.33,111.53 224.56,111.53 U$2.6 218.99,111.12 217.72,112.39 215.35,112.39 214.08,111.12 U$27.6 191.13,111.12 189.87,109.86 187.41,109.86 186.14,108.58 IC17.7
  Bottom 0.508: v229.87,151.76 v229.87,112.39
A2_B  (via drill 0.35)
  Top 0.508: U$26.6 214.08,69.22 215.35,70.48 217.72,70.48 218.99,69.22 U$4.6 224.56,69.62 225.7,69.62 226.56,70.48 v230.5,70.48 | v230.5,29.84 226.56,29.84 225.7,28.98 224.56,28.98 U$3.6 218.99,28.57 217.72,29.84 215.35,29.84 214.08,28.57 U$25.6 191.13,28.57 189.87,27.3 187.41,27.3 186.14,26.04 IC21.7
  Bottom 0.508: v230.5,70.48 v230.5,29.84
A3_A  (via drill 0.35)
  Top 0.508: U$28.5 214.08,153.03 215.35,154.31 217.72,154.31 218.99,153.03 U$1.5 224.56,153.44 226.33,153.44 227.2,154.31 v227.33,154.31 | v227.33,114.94 227.2,114.94 226.33,114.07 224.56,114.07 U$2.5 218.99,113.67 217.72,114.94 215.35,114.94 214.08,113.67 U$27.5 200.02,113.67 198.75,114.94 187.41,114.94 186.14,116.2 IC17.4
  Bottom 0.508: v227.33,154.31 v227.33,114.94
A3_B  (via drill 0.35)
  Top 0.508: U$26.5 214.08,71.75 215.35,73.03 217.72,73.03 218.99,71.75 U$4.5 224.56,72.16 225.7,72.16 226.56,73.03 v227.96,73.03 | v227.96,32.38 226.56,32.38 225.7,31.52 224.56,31.52 U$3.5 218.99,31.11 217.72,32.38 215.35,32.38 214.08,31.11 U$25.5 200.02,32.38 187.41,32.38 186.14,33.66 IC21.4
  Bottom 0.508: v227.96,73.03 v227.96,32.38
A4_A  (via drill 0.35)
  Top 0.508: U$1.4 218.99,155.57 217.72,156.84 215.35,156.84 214.08,155.57 v210.19,155.57 U$28.4 199.39,155.57 195.43,151.61 195.43,147.3 185.92,137.79 164.46,137.79 IC16.7 | U$27.4 v210.19,116.2 214.08,116.2 215.35,117.47 217.72,117.47 218.99,116.2 U$2.4
  Bottom 0.508: v210.19,155.57 v210.19,116.2
A4_B  (via drill 0.35)
  Top 0.508: U$4.4 218.99,74.3 217.72,75.56 215.35,75.56 214.08,74.3 v210.19,74.3 U$26.4 199.39,74.3 195.35,70.26 195.35,65.94 187.19,57.78 169.63,57.78 168.36,56.52 IC20.7 | U$25.4 v210.19,33.66 214.08,33.66 215.35,34.92 217.72,34.92 218.99,33.66 U$3.4
  Bottom 0.508: v210.19,74.3 v210.19,33.66
A5_A  (via drill 0.35)
  Top 0.508: U$1.3 218.99,158.12 217.72,159.38 215.35,159.38 214.08,158.12 v207.64,158.12 U$28.3 198.08,158.12 192.43,152.46 192.43,149.33 188.6,145.5 IC15.9 | U$27.3 v207.64,118.75 214.08,118.75 215.35,120.02 217.72,120.02 218.99,118.75 U$2.3
  Bottom 0.508: v207.64,158.12 v207.64,118.75
A5_B  (via drill 0.35)
  Top 0.508: U$4.3 218.99,76.83 217.72,78.11 215.35,78.11 214.08,76.83 v207.64,76.83 U$26.3 198.12,76.83 192.4,71.12 192.4,67.94 IC19.9 | U$25.3 v207.64,36.2 214.08,36.2 215.35,37.47 217.72,37.47 218.99,36.2 U$3.3
  Bottom 0.508: v207.64,76.83 v207.64,36.2
A6_A  (via drill 0.35)
  Top 0.508: U$1.2 218.99,160.66 217.72,161.93 215.35,161.93 214.08,160.66 v205.11,160.66 U$28.2 196.85,160.66 189.23,153.03 IC15.12 | U$27.2 v205.11,121.28 214.08,121.28 215.35,122.56 217.72,122.56 218.99,121.28 U$2.2
  Bottom 0.508: v205.11,160.66 v205.11,121.28
A6_B  (via drill 0.35)
  Top 0.508: U$26.2 v205.11,79.38 214.08,79.38 215.35,80.64 217.72,80.64 218.99,79.38 U$4.2 | U$25.2 v205.11,38.73 214.08,38.73 215.35,40.01 217.72,40.01 218.99,38.73 U$3.2 | 200.66,79.38 U$26.2 | U$26.2 196.85,79.38 189.23,71.75 IC19.12
  Bottom 0.508: v205.11,79.38 v205.11,38.73
A7_A  (via drill 0.35)
  Top 0.508: U$1.1 218.99,163.19 217.72,164.47 215.35,164.47 214.08,163.19 v203.83,163.19 U$28.1 197.4,163.19 193.59,159.38 184.79,159.38 IC15.4 | U$27.1 v203.83,123.83 214.08,123.83 215.35,125.09 217.72,125.09 218.99,123.83 U$2.1
  Bottom 0.508: v203.83,123.83 v203.83,163.19
A7_B  (via drill 0.35)
  Top 0.508: U$4.1 218.99,81.92 217.72,83.19 215.35,83.19 214.08,81.92 v203.83,81.92 U$26.1 197.49,81.92 193.68,78.11 184.79,78.11 IC19.4 | U$25.1 v203.83,41.27 214.08,41.27 215.35,42.55 217.72,42.55 218.99,41.27 U$3.1
  Bottom 0.508: v203.83,41.27 v203.83,81.92
A8_A  (via drill 0.35)
  Top 0.508: U$2.23 226.61,121.28 225.34,120.02 219.04,120.02 217.77,121.28 U$27.23 216.13,120.88 214.99,120.88 214.13,120.02 v206.38,120.02 | U$1.23 226.61,160.66 225.34,159.38 219.04,159.38 217.77,160.66 U$28.23 216.13,160.25 214.99,160.25 214.13,159.38 v206.38,159.38 197.45,159.38 189.83,151.76 184.79,151.76 IC15.7
  Bottom 0.508: v206.38,120.02 v206.38,159.38
A8_B  (via drill 0.35)
  Top 0.508: U$4.23 226.61,79.38 225.34,78.11 219.04,78.11 217.77,79.38 U$26.23 216.13,78.97 214.99,78.97 214.13,78.11 v206.38,78.11 197.49,78.11 189.87,70.48 184.79,70.48 IC19.7 | U$3.23 226.61,38.73 225.34,37.47 219.04,37.47 217.77,38.73 U$25.23 216.13,38.33 214.99,38.33 214.13,37.47 v206.38,37.47
  Bottom 0.508: v206.38,37.47 v206.38,78.11
A9_A  (via drill 0.35)
  Top 0.508: U$2.22 226.61,118.75 225.34,117.47 219.04,117.47 217.77,118.75 U$27.22 216.13,118.34 214.99,118.34 214.13,117.47 v208.92,117.47 | U$1.22 226.61,158.12 225.34,156.84 219.04,156.84 217.77,158.12 U$28.22 215.3,158.12 214.03,156.84 v208.92,156.84 198.75,156.84 193.93,152.02 193.93,148.29 187.24,141.6 IC16.12
  Bottom 0.508: v208.92,117.47 v208.92,156.84
A9_B  (via drill 0.35)
  Top 0.508: U$4.22 226.61,76.83 225.34,75.56 219.04,75.56 217.77,76.83 U$26.22 216.13,76.43 214.99,76.43 214.13,75.56 v208.92,75.56 198.84,75.56 193.9,70.63 193.9,66.99 188.51,61.59 IC20.12 | U$3.22 226.61,36.2 225.34,34.92 219.04,34.92 217.77,36.2 U$25.22 216.13,35.79 214.99,35.79 214.13,34.92 v208.92,34.92
  Bottom 0.508: v208.92,34.92 v208.92,75.56
A10_A  (via drill 0.35)
  Top 0.508: U$2.19 v231.14,111.12 227.25,111.12 225.98,109.86 219.04,109.86 217.77,111.12 U$27.19 215.3,111.12 214.03,109.86 197.49,109.86 193.68,106.05 IC17.9 | U$28.19 217.77,150.5 219.04,149.22 225.98,149.22 227.25,150.5 v231.14,150.5 U$1.19
  Bottom 0.508: v231.14,111.12 v231.14,150.5
A10_B  (via drill 0.35)
  Top 0.508: U$26.19 217.77,69.22 219.04,67.94 225.34,67.94 226.61,69.22 v231.77,69.22 U$4.19 | U$3.19 v231.77,28.57 226.61,28.57 225.34,27.3 219.04,27.3 217.77,28.57 U$25.19 216.13,28.17 214.99,28.17 214.13,27.3 197.49,27.3 193.68,23.5 IC21.9
  Bottom 0.508: v231.77,28.57 v231.77,69.22
CS_A  (via drill 0.35)  (1 unrouted)
  Top 0.508: 216.13,108.18 U$27.18 215.3,108.58 214.03,107.31 v212.73,107.31 198.66,107.31 191.04,99.69 164.46,99.69 IC18.7 | U$28.18 216.13,147.55 214.99,147.55 214.13,146.69 v212.73,146.69
  Bottom 0.508: v212.73,146.69 v212.73,107.31
CS_B  (via drill 0.35)  (1 unrouted)
  Top 0.508: U$26.18 216.13,66.27 214.99,66.27 214.13,65.41 v212.73,65.41 201.3,65.41 | U$25.18 216.13,25.63 214.99,25.63 214.13,24.77 v212.73,24.77 198.75,24.77 191.13,17.14 164.46,17.14 IC22.7
  Bottom 0.508: v212.73,65.41 v212.73,24.77
CSIN  (2 unrouted)
D0  (1 unrouted)
D1  (1 unrouted)
D2  (1 unrouted)
D3  (1 unrouted)
D4  (1 unrouted)
D5  (1 unrouted)
D6  (1 unrouted)
D7  (1 unrouted)
D8  (1 unrouted)
D9  (1 unrouted)
D10  (1 unrouted)
D11  (1 unrouted)
D12  (1 unrouted)
D13  (1 unrouted)
D14  (1 unrouted)
D15  (1 unrouted)
D16  (1 unrouted)
D17  (1 unrouted)
D18  (1 unrouted)
FRAMECOMPLETE  (2 unrouted)
GND  (26 unrouted)
  Top 2.032: P2.22 4.83,48.9 P2.21 | P1.Z 305.05,48.9 P1.Y
  Top 5.08: 4.83,48.9 10.16,48.9 13.97,45.09 13.97,3.81 295.91,3.81 295.91,45.09 299.72,48.9 305.05,48.9
  Bottom 1.016: IC22.8 160.65,13.34 | 160.65,13.34 160.65,3.81 | U$25.12 198.75,13.34 | 198.75,3.81 198.75,13.34 | IC21.8 178.44,23.5 | 178.44,3.81 178.44,23.5 | U$3.12 221.62,13.34 | 221.62,3.81 221.62,13.34 | IC13.10 249.56,15.88 | 249.56,15.88 249.56,3.81 249.56,3.17 | IC10.10 266.06,15.88 | 266.06,15.88 266.06,3.81 | 266.06,15.88 266.06,56.52 | 266.06,56.52 266.06,88.9 | 266.06,88.9 266.06,98.42 | 266.06,98.42 266.06,137.79 IC4.10 | 266.06,98.42 IC6.10 | 266.06,88.9 C10.2 | 266.06,56.52 IC8.10 | 249.56,15.88 249.56,56.52 | 249.56,56.52 249.56,88.9 | 249.56,88.9 249.56,98.42 | 249.56,98.42 249.56,137.79 IC5.10 | 249.56,98.42 IC7.10 | IC9.10 249.56,56.52 | 221.62,13.34 221.62,53.98 | 221.62,53.98 221.62,88.9 | 221.62,88.9 221.62,95.89 | 221.62,95.89 221.62,135.25 U$1.12 | 221.62,95.89 U$2.12 | 221.62,53.98 U$4.12 | 198.75,13.34 198.75,53.98 | 198.75,53.98 198.75,88.9 | 198.75,88.9 198.75,95.89 | 198.75,95.89 198.75,135.25 U$28.12 | 198.75,95.89 U$27.12 | 198.75,53.98 U$26.12 | 178.44,23.5 178.44,64.14 | 178.44,64.14 178.44,88.9 | 178.44,88.9 178.44,106.05 | 178.44,106.05 178.44,145.41 IC15.8 | 178.44,106.05 IC17.8 | 178.44,64.14 IC19.8 | 160.65,13.34 160.65,53.98 | 160.65,53.98 160.65,88.9 | 160.65,88.9 160.65,95.89 | 160.65,95.89 160.65,133.99 IC16.8 | 160.65,95.89 IC18.8 | 160.65,53.98 IC20.8 | 249.56,88.9 C9.2 | C8.2 221.62,88.9 | C7.2 198.75,88.9 | C6.2 178.44,88.9 | C5.2 160.65,88.9 | U1.8 123.83,13.34 | 123.83,13.34 123.83,3.81 | 123.83,13.34 123.83,38.73 | 123.83,38.73 123.83,64.14 | U3.8 123.83,64.14 | 123.83,38.73 U2.8 | U4.8 106.05,13.34 | 106.05,13.34 106.05,3.81 | 106.05,13.34 106.05,40.01 | 106.05,40.01 106.05,65.41 IC42.7 | IC59.7 106.05,40.01 | 123.83,64.14 123.83,87 C4.2 131.44,90.81 131.44,102.26 129.59,104.12 129.59,106.7 131.44,108.56 131.44,110.49
  Bottom 1.016: IC34.7 88.27,40.01 | 88.27,40.01 88.27,4.45 88.9,3.81 | 88.27,40.01 88.27,65.41 | 88.27,65.41 IC14.7 | 88.27,65.41 88.27,87 | 88.27,87 C3.2 | B1.GND@4 62.61,161.04 62.87,161.29 | 131.44,110.49 B1.GND@2 | 131.44,110.49 B1.GND@3 | B1.GND@0 B1.GND@1 80.11,104.67 80.11,104.66 88.27,96.51 88.27,87
  Bottom 2.032: P2.22 4.83,48.9 P2.21 | P1.Z 305.05,48.9 P1.Y
  Bottom 2.54: X1.2 57.08,161.37 57.15,161.29 | 57.15,161.29 62.87,161.29 65.41,161.29 65.41,165.96 X1.4 | 57.15,161.29 41.27,161.29 36.83,156.84 36.83,4.45 37.47,3.81
  Bottom 5.08: 4.83,48.9 10.16,48.9 13.97,45.09 13.97,3.81 37.47,3.81 88.9,3.81 106.05,3.81 123.83,3.81 160.65,3.81 178.44,3.81 198.75,3.81 221.62,3.81 249.56,3.81 266.06,3.81 295.91,3.81 295.91,45.09 299.72,48.9 305.05,48.9
N$2  (1 unrouted)
N$5  (1 unrouted)
N$6  (1 unrouted)
N$48  (1 unrouted)
  Top 0.508: IC34.1 R1.2 83.71,55.24 82.44,56.52 69.98,56.52 Q1.1
N$52  (2 unrouted)
  Top 0.508: IC34.5 R1.1
  Bottom 0.508: C2.1 81.28,47.62 R1.1
N$61
  Top 0.508: IC34.3 84.45,50.16 R2.2 76.83,55.24 C2.2
N$69
  Top 0.508: Q1.2 72.39,42.67 C1.1
N$74
  Top 0.508: IC34.4 81.92,47.62 R2.1 77.47,45.09 C1.2
OE_A  (via drill 0.35)
  Top 0.508: U$2.20 v228.6,113.67 227.25,113.67 225.98,112.39 219.04,112.39 217.77,113.67 U$27.20 216.13,113.26 214.99,113.26 214.13,112.39 199.39,112.39 198.12,113.67 IC17.12 | U$28.20 217.77,153.03 219.04,151.76 225.98,151.76 227.25,153.03 v228.6,153.03 U$1.20
  Bottom 0.508: v228.6,113.67 v228.6,153.03
OE_B  (via drill 0.35)
  Top 0.508: U$26.20 217.77,71.75 219.04,70.48 225.34,70.48 226.61,71.75 v229.24,71.75 U$4.20 | U$3.20 v229.24,31.11 226.61,31.11 225.34,29.84 219.04,29.84 217.77,31.11 U$25.20 216.13,30.71 214.99,30.71 214.13,29.84 200.02,29.84 198.75,31.11 IC21.12
  Bottom 0.508: v229.24,31.11 v229.24,71.75
OEIN  (2 unrouted)
P  (via drill 0.35)  (10 unrouted)
  Top 0.508: R3.2 122.56,41.27 U2.7 128.91,41.27 v130.18,40.01 131.44,38.73 U2.9 | U3.9 131.44,64.14 v130.18,65.41 128.91,66.67 U3.7 | U1.9 131.44,13.34 v130.18,14.61 128.91,15.88 U1.7
  Bottom 0.508: v130.18,14.61 v130.18,40.01 v130.18,65.41
PORTF0  (1 unrouted)
PORTF1  (1 unrouted)
PORTF2  (1 unrouted)
PORTF3  (1 unrouted)
PORTF4  (1 unrouted)
PORTF5  (1 unrouted)
PORTF6  (1 unrouted)
PORTF7  (1 unrouted)
PORTK0  (1 unrouted)
PORTK1  (1 unrouted)
PORTK2  (1 unrouted)
PORTK3  (1 unrouted)
PORTK4  (1 unrouted)
PORTK5  (1 unrouted)
PORTK6  (1 unrouted)
PORTK7  (1 unrouted)
PROCESSOROVERRIDE  (2 unrouted)
PROCESSORREADY  (1 unrouted)
RESETVRAMPC  (1 unrouted)
VCC
  Top 1.016: 136.53,94.61 136.53,87 C4.1 | C3.1 97.16,94.61
  Top 2.032: P2.A 4.83,128.91 P2.B | P1.1 305.05,128.91 P1.2
  Top 2.54: 45.09,173.99 45.09,102.23 52.7,94.61 97.16,94.61 136.53,94.61 | X1.1 53.12,173.76 53.34,173.99
  Top 5.08: 4.83,128.91 10.16,128.91 13.97,132.72 13.97,173.99 45.09,173.99 53.34,173.99 295.91,173.99 295.91,132.72 299.72,128.91 305.05,128.91
  Bottom 1.016: IC16.16 173.36,151.76 | 173.36,173.99 173.36,151.76 | IC15.16 191.13,163.19 | 191.13,163.19 191.13,172.72 189.87,173.99 | U$28.24 219.07,163.19 | 219.07,173.99 219.07,163.19 | U$1.24 241.94,163.19 | 241.94,173.99 241.94,163.19 | IC5.20 262.25,160.66 | 262.25,173.99 262.25,160.66 | IC4.20 278.76,160.66 | 278.76,173.99 278.76,160.66 | 173.36,151.76 173.36,113.67 | 173.36,113.67 173.36,88.9 | 173.36,88.9 173.36,71.75 | 173.36,71.75 173.36,31.11 IC22.16 | IC20.16 173.36,71.75 | IC18.16 173.36,113.67 | 191.13,163.19 191.13,123.83 | 191.13,123.83 191.13,88.9 | 191.13,88.9 191.13,81.92 | 191.13,81.92 191.13,41.27 IC21.16 | IC19.16 191.13,81.92 | IC17.16 191.13,123.83 | 219.07,163.19 219.07,123.83 | 219.07,123.83 219.07,88.9 | 219.07,88.9 219.07,81.92 | 219.07,81.92 219.07,41.27 U$25.24 | U$26.24 219.07,81.92 | U$27.24 219.07,123.83 | 241.94,163.19 241.94,123.83 | 241.94,123.83 241.94,88.9 | 241.94,88.9 241.94,81.92 | 241.94,81.92 241.94,41.27 U$3.24 | U$4.24 241.94,81.92 | U$2.24 241.94,123.83 | 262.25,160.66 262.25,121.28 | 262.25,121.28 262.25,88.9 | 262.25,88.9 262.25,79.38 | 262.25,79.38 262.25,38.73 IC13.20 | 278.76,160.66 278.76,121.28 | 278.76,121.28 278.76,88.9 | 278.76,88.9 278.76,79.38 | 278.76,79.38 278.76,38.73 IC10.20 | C9.1 262.25,88.9 | C10.1 278.76,88.9 | C8.1 241.94,88.9 | C7.1 219.07,88.9 | C6.1 191.13,88.9 | C5.1 173.36,88.9 | IC9.20 262.25,79.38 | IC8.20 278.76,79.38 | IC7.20 262.25,121.28 | IC6.20 278.76,121.28 | C4.1 136.53,87 136.53,81.92 | 136.53,81.92 U3.16 | 136.53,81.92 136.53,56.52 | 136.53,56.52 136.53,31.11 U1.16 | U2.16 136.53,56.52 | 118.75,55.24 118.75,31.11 U4.16 | 118.75,80.64 118.75,55.24 | 118.75,80.64 118.75,87 100.97,87 | 118.75,80.64 IC42.14
  Bottom 1.016: 100.97,87 C3.1 | IC59.14 118.75,55.24 | 118.75,55.24 R3.1 | IC34.14 100.97,55.24 100.97,80.64 | 100.97,80.64 100.97,87 | IC14.14 100.97,80.64
  Bottom 2.032: P2.B 4.83,128.91 P2.A | P1.1 305.05,128.91 P1.2
  Bottom 2.54: X1.1 53.12,173.76 53.34,173.99
  Bottom 5.08: 4.83,128.91 10.16,128.91 13.97,132.72 13.97,173.99 53.34,173.99 173.36,173.99 189.87,173.99 219.07,173.99 241.94,173.99 262.25,173.99 278.76,173.99 295.91,173.99 295.91,132.72 299.72,128.91 305.05,128.91
VPC0  (2 unrouted)
VPC1  (2 unrouted)
VPC2  (2 unrouted)
VPC3  (2 unrouted)
VPC4  (2 unrouted)
VPC5  (2 unrouted)
VPC6  (2 unrouted)
VPC7  (2 unrouted)
VPC8  (2 unrouted)
VPC9  (2 unrouted)
VPC10  (2 unrouted)
VPC11  (2 unrouted)
VRAM0  (2 unrouted)
VRAM1  (2 unrouted)
VRAM2  (2 unrouted)
VRAM3  (2 unrouted)
VRAM4  (2 unrouted)
VRAM5  (2 unrouted)
VRAM6  (2 unrouted)
VRAM7  (2 unrouted)
VRAM8  (2 unrouted)
VRAM9  (2 unrouted)
VRAM10  (2 unrouted)
VRAM11  (2 unrouted)
VRAM12  (2 unrouted)
VRAM13  (2 unrouted)
VRAM14  (2 unrouted)
VRAM15  (2 unrouted)
VRAM_A_0
  Top 0.508: U$27.9 214.08,103.5 215.35,104.78 217.72,104.78 218.99,103.5 U$2.9 224.56,103.91 225.7,103.91 226.56,104.78 240.67,104.78 250.82,114.94 253.37,114.94 254.63,116.2 IC7.18 IC6.3
VRAM_A_1
  Top 0.508: U$27.10 214.08,100.97 215.35,102.23 217.72,102.23 218.99,100.97 U$2.10 224.56,101.37 225.7,101.37 226.56,102.23 243.29,102.23 250.91,109.86 253.37,109.86 254.63,111.12 IC7.16 IC6.5
VRAM_A_2
  Top 0.508: U$27.11 214.08,98.42 215.35,99.69 217.72,99.69 218.99,98.42 U$2.11 224.56,98.83 225.7,98.83 226.56,99.69 245.83,99.69 250.91,104.78 253.37,104.78 254.63,106.05 IC7.14 IC6.7
VRAM_A_3
  Top 0.508: U$27.13 221.7,95.89 222.97,94.61 225.34,94.61 226.61,95.89 U$2.13 247.01,95.89 250.82,99.69 253.28,99.69 254.55,100.97 IC7.12 IC6.9
VRAM_A_4
  Top 0.508: U$27.14 217.77,98.42 219.04,97.16 225.34,97.16 226.61,98.42 U$2.14 247.1,98.42 250.91,102.23 253.37,102.23 254.63,103.5 IC7.13 IC6.8
VRAM_A_5
  Top 0.508: U$27.15 217.77,100.97 219.04,99.69 225.34,99.69 226.61,100.97 U$2.15 244.56,100.97 250.91,107.31 253.37,107.31 254.63,108.58 IC7.15 IC6.6
VRAM_A_6
  Top 0.508: U$27.16 217.77,103.5 219.04,102.23 225.34,102.23 226.61,103.5 U$2.16 241.94,103.5 250.82,112.39 253.28,112.39 254.55,113.67 IC7.17 IC6.4
VRAM_A_7
  Top 0.508: U$27.17 217.77,106.05 219.04,104.78 225.34,104.78 226.61,106.05 U$2.17 250.82,117.47 253.37,117.47 254.63,118.75 IC7.19 IC6.2
VRAM_A_8
  Top 0.508: U$28.9 214.08,142.88 215.35,144.15 217.72,144.15 218.99,142.88 U$1.9 224.56,143.28 226.33,143.28 227.2,144.15 240.67,144.15 250.82,154.31 253.28,154.31 254.55,155.57 IC5.18 IC4.3
VRAM_A_9
  Top 0.508: U$28.10 214.08,140.34 215.35,141.6 217.72,141.6 218.99,140.34 U$1.10 224.56,140.74 226.33,140.74 227.2,141.6 243.29,141.6 250.91,149.22 253.37,149.22 254.63,150.5 IC5.16 IC4.5
VRAM_A_10
  Top 0.508: U$28.11 214.08,137.79 215.35,139.06 217.72,139.06 218.99,137.79 U$1.11 224.56,138.2 226.33,138.2 227.2,139.06 245.75,139.06 250.82,144.15 253.28,144.15 254.55,145.41 IC5.14 IC4.7
VRAM_A_11
  Top 0.508: U$28.13 221.7,135.25 222.97,133.99 225.98,133.99 227.25,135.25 U$1.13 247.01,135.25 250.82,139.06 253.28,139.06 254.55,140.34 IC5.12 IC4.9
VRAM_A_12
  Top 0.508: U$28.14 217.77,137.79 219.04,136.53 225.98,136.53 227.25,137.79 U$1.14 247.01,137.79 250.82,141.6 253.28,141.6 254.55,142.88 IC5.13 IC4.8
VRAM_A_13
  Top 0.508: U$28.15 217.77,140.34 219.04,139.06 225.98,139.06 227.25,140.34 U$1.15 244.48,140.34 250.82,146.69 253.28,146.69 254.55,147.96 IC5.15 IC4.6
VRAM_A_14
  Top 0.508: U$28.16 217.77,142.88 219.04,141.6 225.98,141.6 227.25,142.88 U$1.16 242.02,142.88 250.91,151.76 253.37,151.76 254.63,153.03 IC5.17 IC4.4
VRAM_A_15
  Top 0.508: U$28.17 217.77,145.41 219.04,144.15 225.98,144.15 227.25,145.41 U$1.17 250.82,156.84 253.28,156.84 254.55,158.12 IC5.19 IC4.2
VRAM_B_0
  Top 0.508: U$25.9 214.08,20.95 215.35,22.23 217.72,22.23 218.99,20.95 U$3.9 224.56,21.36 225.7,21.36 226.56,22.23 240.75,22.23 250.91,32.38 253.37,32.38 254.63,33.66 IC13.18 IC10.3
VRAM_B_1
  Top 0.508: U$25.10 214.08,18.41 215.35,19.68 217.72,19.68 218.99,18.41 U$3.10 224.56,18.82 225.7,18.82 226.56,19.68 243.29,19.68 250.91,27.3 253.37,27.3 254.63,28.57 IC13.16 IC10.5
VRAM_B_2
  Top 0.508: U$25.11 214.08,15.88 215.35,17.14 217.72,17.14 218.99,15.88 U$3.11 224.56,16.28 225.7,16.28 226.56,17.14 245.75,17.14 250.82,22.23 253.28,22.23 254.55,23.5 IC13.14 IC10.7
VRAM_B_3
  Top 0.508: U$25.13 221.7,13.34 222.97,12.06 225.34,12.06 226.61,13.34 U$3.13 247.01,13.34 250.82,17.14 253.28,17.14 254.55,18.41 IC13.12 IC10.9
VRAM_B_4
  Top 0.508: U$25.14 217.77,15.88 219.04,14.61 225.34,14.61 226.61,15.88 U$3.14 247.01,15.88 250.82,19.68 253.28,19.68 254.55,20.95 IC13.13 IC10.8
VRAM_B_5
  Top 0.508: U$25.15 217.77,18.41 219.04,17.14 225.34,17.14 226.61,18.41 U$3.15 244.48,18.41 250.82,24.77 253.28,24.77 254.55,26.04 IC13.15 IC10.6
VRAM_B_6
  Top 0.508: U$25.16 217.77,20.95 219.04,19.68 225.34,19.68 226.61,20.95 U$3.16 241.94,20.95 250.82,29.84 253.28,29.84 254.55,31.11 IC13.17 IC10.4
VRAM_B_7
  Top 0.508: U$25.17 217.77,23.5 219.04,22.23 225.34,22.23 226.61,23.5 U$3.17 250.82,34.92 253.28,34.92 254.55,36.2 IC13.19 IC10.2
VRAM_B_8
  Top 0.508: U$26.9 214.08,61.59 215.35,62.87 217.72,62.87 218.99,61.59 U$4.9 224.56,62 225.7,62 226.56,62.87 240.67,62.87 250.82,73.03 253.37,73.03 254.63,74.3 IC9.18 IC8.3
VRAM_B_9
  Top 0.508: U$26.10 214.08,59.05 215.35,60.33 217.72,60.33 218.99,59.05 U$4.10 224.56,59.46 225.7,59.46 226.56,60.33 243.2,60.33 250.82,67.94 253.28,67.94 254.55,69.22 IC9.16 IC8.5
VRAM_B_10
  Top 0.508: U$26.11 214.08,56.52 215.35,57.78 217.72,57.78 218.99,56.52 U$4.11 224.56,56.92 225.7,56.92 226.56,57.78 245.75,57.78 250.82,62.87 253.37,62.87 254.63,64.14 IC9.14 IC8.7
VRAM_B_11  (1 unrouted)
  Top 0.508: U$4.13 247.01,53.98 250.82,57.78 253.28,57.78 254.55,59.05 IC9.12 IC8.9
VRAM_B_12
  Top 0.508: U$26.14 217.77,56.52 219.04,55.24 225.34,55.24 226.61,56.52 U$4.14 247.1,56.52 250.91,60.33 253.37,60.33 254.63,61.59 IC9.13 IC8.8
VRAM_B_13
  Top 0.508: U$26.15 217.77,59.05 219.04,57.78 225.34,57.78 226.61,59.05 U$4.15 244.56,59.05 250.91,65.41 253.37,65.41 254.63,66.67 IC9.15 IC8.6
VRAM_B_14
  Top 0.508: U$26.16 217.77,61.59 219.04,60.33 225.34,60.33 226.61,61.59 U$4.16 241.94,61.59 250.82,70.48 253.37,70.48 254.63,71.75 IC9.17 IC8.4
VRAM_B_15
  Top 0.508: U$26.17 217.77,64.14 219.04,62.87 225.34,62.87 226.61,64.14 U$4.17 250.82,75.56 253.37,75.56 254.63,76.83 IC9.19 IC8.2
VRAMA0  (2 unrouted)
VRAMA1  (2 unrouted)
VRAMA2  (2 unrouted)
VRAMA3  (2 unrouted)
VRAMA4  (2 unrouted)
VRAMA5  (2 unrouted)
VRAMA6  (2 unrouted)
VRAMA7  (2 unrouted)
VRAMA8  (2 unrouted)
VRAMA9  (2 unrouted)
VRAMA10  (2 unrouted)
VRAMBANKSELECT  (12 unrouted)
VRAMIN0  (2 unrouted)
VRAMIN1  (2 unrouted)
VRAMIN2  (2 unrouted)
VRAMIN3  (2 unrouted)
VRAMIN4  (2 unrouted)
VRAMIN5  (2 unrouted)
VRAMIN6  (2 unrouted)
VRAMIN7  (2 unrouted)
VRAMIN8  (2 unrouted)
VRAMIN9  (2 unrouted)
VRAMIN10  (2 unrouted)
VRAMIN11  (2 unrouted)
VRAMIN12  (2 unrouted)
VRAMIN13  (2 unrouted)
VRAMIN14  (2 unrouted)
VRAMIN15  (2 unrouted)
VRAMPC  (3 unrouted)
WE_A  (via drill 0.35)
  Top 0.508: U$2.21 226.61,116.2 225.34,114.94 219.04,114.94 217.77,116.2 U$27.21 216.13,115.8 214.99,115.8 214.13,114.94 v211.45,114.94 | U$1.21 226.61,155.57 225.34,154.31 219.04,154.31 217.77,155.57 U$28.21 216.13,155.17 214.99,155.17 214.13,154.31 v211.45,154.31 200.11,154.31 196.93,151.12 196.93,146.31 184.6,133.99 IC16.9
  Bottom 0.508: v211.45,114.94 v211.45,154.31
WE_B  (via drill 0.35)
  Top 0.508: U$4.21 226.61,74.3 225.34,73.03 219.04,73.03 217.77,74.3 U$26.21 216.13,73.89 214.99,73.89 214.13,73.03 v211.45,73.03 200.11,73.03 197.49,70.4 197.49,65.59 185.87,53.98 IC20.9 | U$3.21 226.61,33.66 225.34,32.38 219.04,32.38 217.77,33.66 U$25.21 216.13,33.25 214.99,33.25 214.13,32.38 v211.45,32.38
  Bottom 0.508: v211.45,32.38 v211.45,73.03
WEIN  (2 unrouted)

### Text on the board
Top: Double-Buffered Vector RAM Board | (C) Kincaid Arcade 6/8/2020 | KincaidArcade.com | Designed By: Alexander K. Haley | (A 17 year old!) | Board and design licensed under CC BY-SA 4.0 | https://creativecommons.org/licenses/by-sa/4.0/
